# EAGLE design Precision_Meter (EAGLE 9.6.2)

## Sheet 1 of 4: ADC, Buff Amp, VREF Circuits
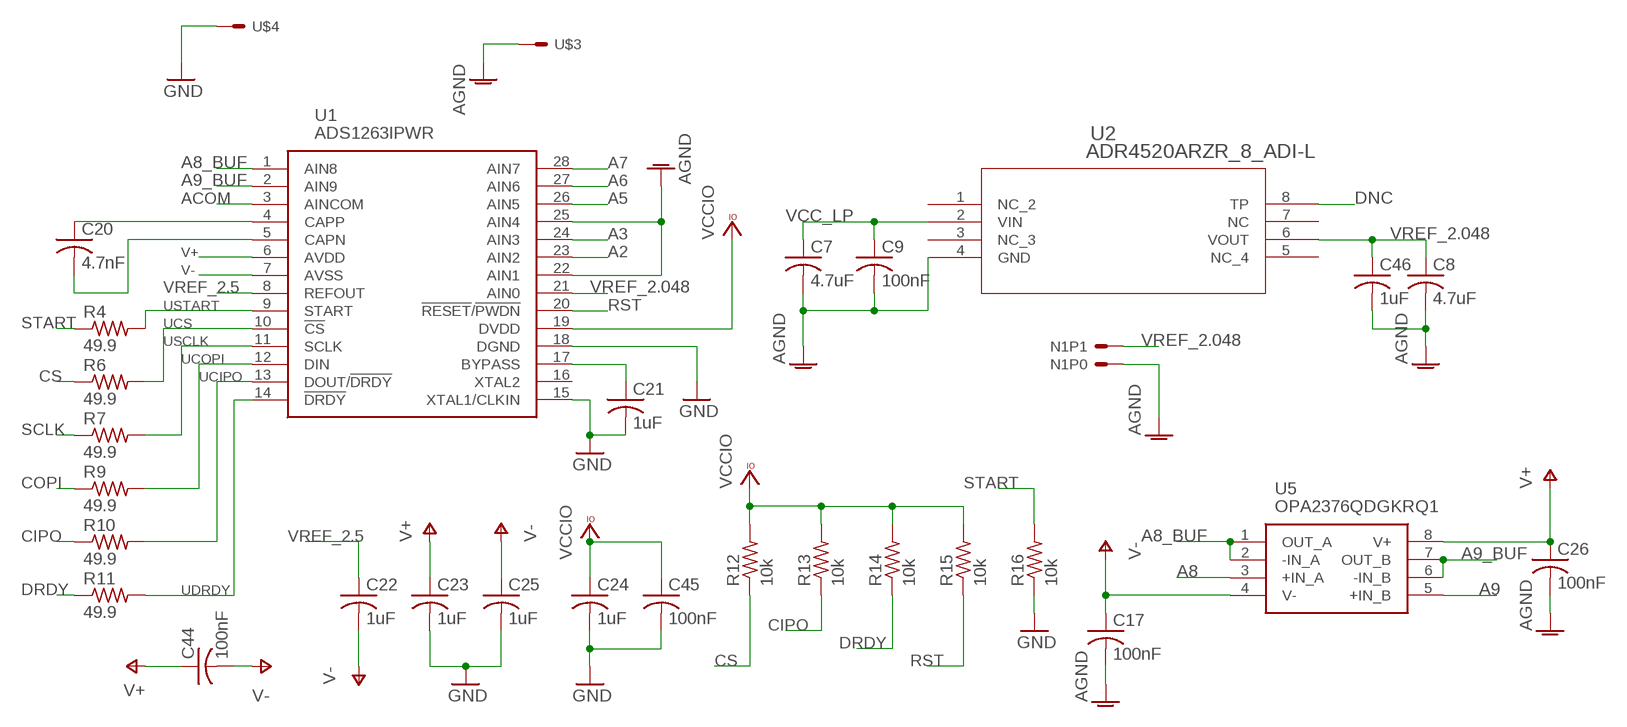
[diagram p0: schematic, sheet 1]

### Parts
C7  4.7uF  C-USC0603  [C0603]
C8  4.7uF  C-USC0603  [C0603]
C9  100nF  C-USC0603  [C0603]
C17  100nF  C-USC0603  [C0603]
C20  4.7nF  C-USC0603  [C0603]
C21  1uF  C-USC0603  [C0603]
C22  1uF  C-USC0603  [C0603]
C23  1uF  C-USC0603  [C0603]
C24  1uF  C-USC0603  [C0603]
C25  1uF  C-USC0603  [C0603]
C26  100nF  C-USC0603  [C0603]
C44  100nF  C-USC0603  [C0603]
C45  100nF  C-USC0603  [C0603]
C46  1uF  C-USC0603  [C0603]
N1  2PINHEADER  [2PINHEADER]
R4  49.9  R-US_R0603  [R0603]
R6  49.9  R-US_R0603  [R0603]
R7  49.9  R-US_R0603  [R0603]
R9  49.9  R-US_R0603  [R0603]
R10  49.9  R-US_R0603  [R0603]
R11  49.9  R-US_R0603  [R0603]
R12  10k  R-US_R0603  [R0603]
R13  10k  R-US_R0603  [R0603]
R14  10k  R-US_R0603  [R0603]
R15  10k  R-US_R0603  [R0603]
R16  10k  R-US_R0603  [R0603]
U1  ADS1263IPWR  [SOP65P640X120-28N]
U2  ADR4520ARZR_8_ADI-L  [R_8_ADI-L]
U5  OPA2376QDGKRQ1  [SOP65P490X110-8N]
U$3  1PINHEADER_S  [1PINHEADER_S]
U$4  1PINHEADER_S  [1PINHEADER_S]

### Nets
A2: U1.23(AIN2) ; also sheet 3
A3: U1.24(AIN3) ; also sheet 3
A5: U1.26(AIN5) ; also sheet 3
A6: U1.27(AIN6) ; also sheet 3
A7: U1.28(AIN7) ; also sheet 3
A8: U5.3(+IN_A) ; also sheet 3
A8_BUF: U1.1(AIN8) U5.1(OUT_A) U5.2(-IN_A)
A9: U5.5(+IN_B) ; also sheet 3
A9_BUF: U1.2(AIN9) U5.6(-IN_B) U5.7(OUT_B)
ACOM: U1.3(AINCOM) ; also sheet 3
AGND: C7.2 C8.2 C9.2 C17.2 C26.2 C46.2 N1.P0 U1.22(AIN1) U1.25(AIN4) U2.4(GND) U$3.P$1(S) ; also sheet 3,4
CIPO: R10.1 R13.1 ; also sheet 3
COPI: R9.1 ; also sheet 3
CS: R6.1 R12.1 ; also sheet 3
DNC: U2.8(TP)
DRDY: R11.1 R14.1 ; also sheet 3
GND: C21.2 C23.2 C24.2 C25.2 C45.2 R16.1 U1.15(XTAL1/CLKIN) U1.18(DGND) U$4.P$1(S) ; also sheet 2,3,4
N$8: C20.1 U1.4(CAPP)
N$9: C20.2 U1.5(CAPN)
N$28: C21.1 U1.17(BYPASS)
RST: R15.1 U1.20(!RESET!/!PWDN) ; also sheet 2,3
SCLK: R7.1 ; also sheet 3
START: R4.1 R16.2 ; also sheet 3
UCIPO: R10.2 U1.13(DOUT/!DRDY)
UCOPI: R9.2 U1.12(DIN)
UCS: R6.2 U1.10(!CS)
UDRDY: R11.2 U1.14(!DRDY)
USCLK: R7.2 U1.11(SCLK)
USTART: R4.2 U1.9(START)
V+: C23.1 C26.1 C44.1 U1.6(AVDD) U5.8(V+) ; also sheet 2
V-: C17.1 C22.2 C25.1 C44.2 U1.7(AVSS) U5.4(V-) ; also sheet 2
VCC_LP: C7.1 C9.1 U2.2(VIN) ; also sheet 2,4
VCCIO: C24.1 C45.1 R12.2 R13.2 R14.2 R15.2 U1.19(DVDD) ; also sheet 2,3
VREF_2.5: C22.1 U1.8(REFOUT)
VREF_2.048: C8.1 C46.1 N1.P1 U1.21(AIN0) U2.6(VOUT)
Unconnected: U1.16(XTAL2) U2.1(NC_2) U2.3(NC_3) U2.5(NC_4) U2.7(NC)

## Sheet 2 of 4: Power Circuits
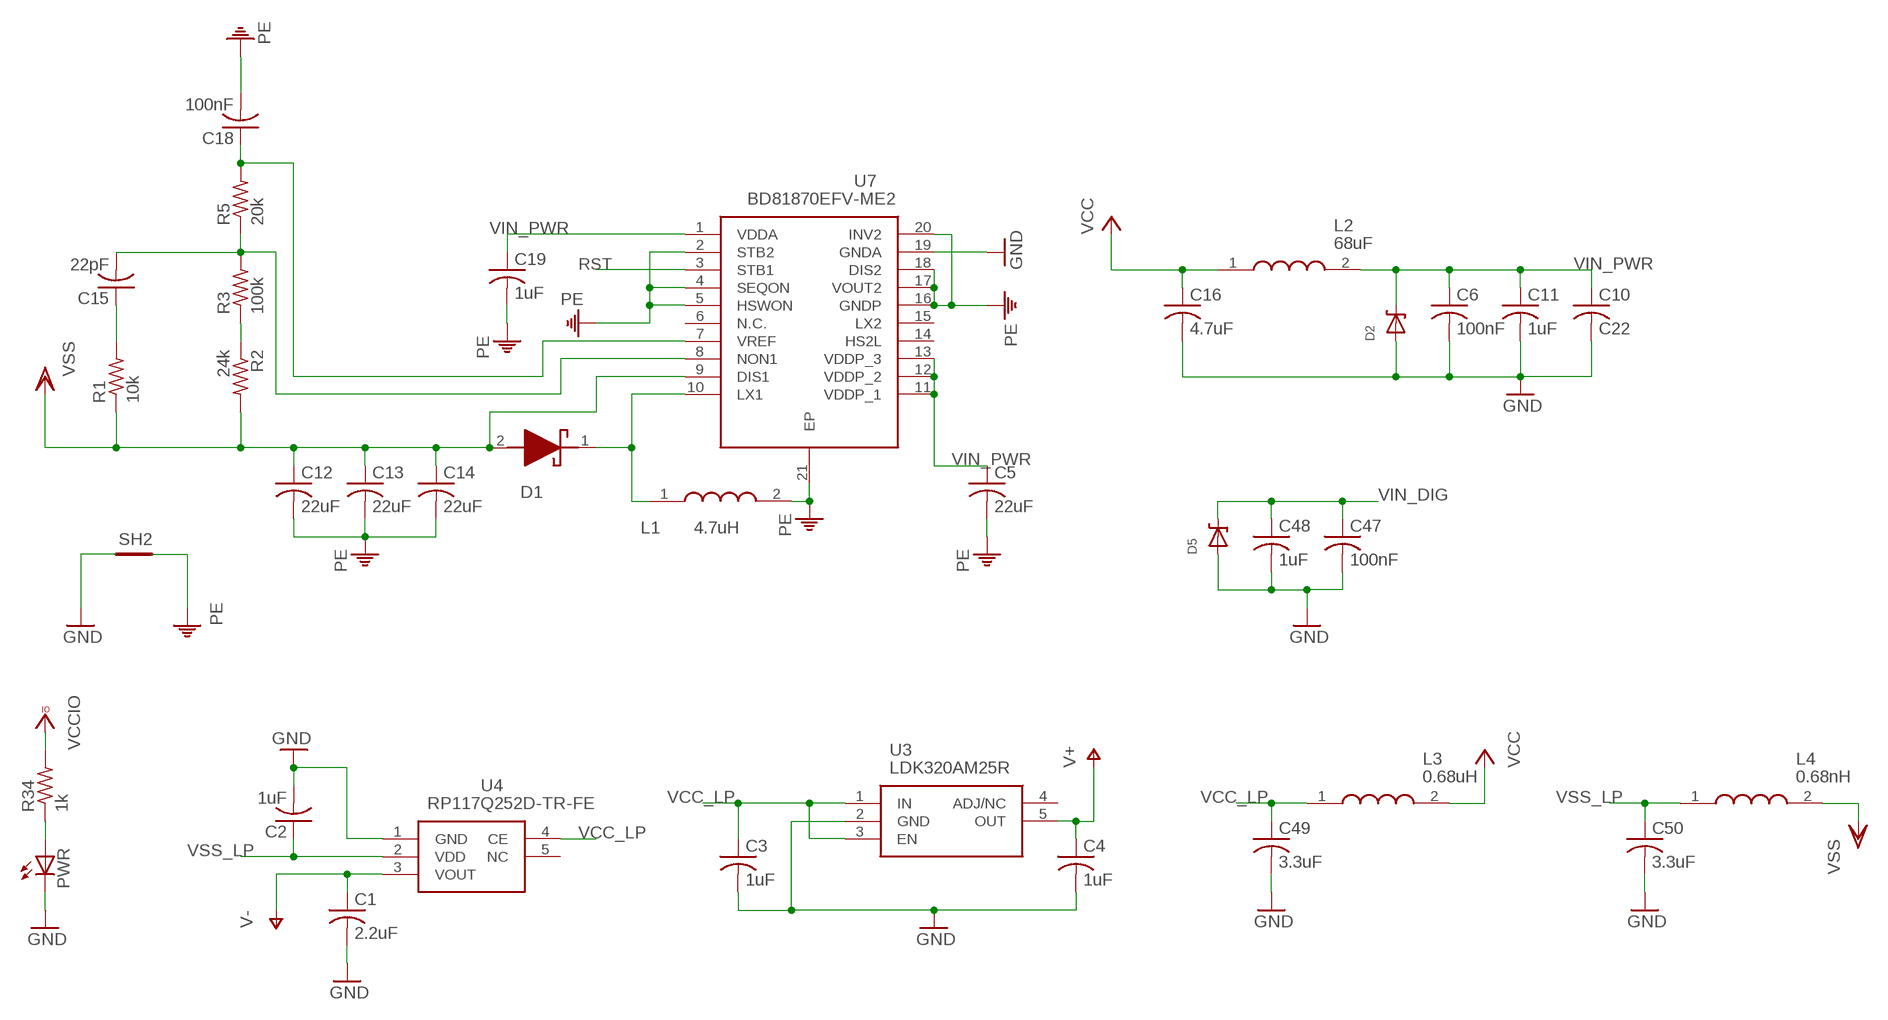
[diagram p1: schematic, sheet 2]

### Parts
C1  2.2uF  C-USC0603  [C0603]
C2  1uF  C-USC0603  [C0603]
C3  1uF  C-USC0603  [C0603]
C4  1uF  C-USC0603  [C0603]
C5  22uF  C-USC0603  [C0603]
C6  100nF  C-USC0603  [C0603]
C10  C22  C-USC0603  [C0603]
C11  1uF  C-USC0603  [C0603]
C12  22uF  C-USC0603  [C0603]
C13  22uF  C-USC0603  [C0603]
C14  22uF  C-USC0603  [C0603]
C15  22pF  C-USC0603  [C0603]
C16  4.7uF  C-USC0603  [C0603]
C18  100nF  C-USC0603  [C0603]
C19  1uF  C-USC0603  [C0603]
C47  100nF  C-USC0603  [C0603]
C48  1uF  C-USC0603  [C0603]
C49  3.3uF  C-USC0603  [C0603]
C50  3.3uF  C-USC0603  [C0603]
D1  RSX051VAM30TR  [RSX051VAM30TR]
D2  DDZ5V6ASF  [DDZ5V6ASF]
D5  DDZ5V6ASF  [DDZ5V6ASF]
L1  4.7uH  LQM21PN4R7MGSD  [LQM21PHR47NG0D]
L2  68uF  LBC3225T680MR  [INDC3225X270N]
L3  0.68uH  MLF2012DR68MT000  [INDC2012X145N]
L4  0.68nH  MLF2012DR68MT000  [INDC2012X145N]
PWR  LEDCHIPLED_0603  [CHIPLED_0603]
R1  10k  R-US_R0603  [R0603]
R2  24k  R-US_R0603  [R0603]
R3  100k  R-US_R0603  [R0603]
R5  20k  R-US_R0603  [R0603]
R34  1k  R-US_R0603  [R0603]
SH2  SHORT-HT5  [SHORT_TOP-50]
U3  LDK320AM25R  [SOT95P280X125-5N]
U4  RP117Q252D-TR-FE  [SOT65P210X110-5N]
U7  BD81870EFV-ME2  [SOP65P640X100-21N]

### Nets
GND: C1.2 C2.2 C3.2 C4.2 C6.2 C10.2 C11.2 C16.2 C47.2 C48.2 C49.2 C50.2 D2.P$1(A) D5.P$1(A) PWR.C SH2.1 U3.2(GND) U4.1(GND) U7.19(GNDA) ; also sheet 1,3,4
N$4: C15.2 R3.2 R5.1 U7.8(NON1)
N$5: D1.1(K) L1.1 U7.10(LX1)
N$6: C18.1 R5.2 U7.7(VREF)
N$7: C15.1 R1.2
N$11: R2.1 R3.1
N$19: PWR.A R34.1
PE: C5.2 C12.2 C13.2 C14.2 C18.2 C19.2 L1.2 SH2.2 U7.2(STB2) U7.4(SEQON) U7.5(HSWON) U7.16(GNDP) U7.17(VOUT2) U7.18(DIS2) U7.20(INV2) U7.21(EP)
RST: U7.3(STB1) ; also sheet 1,3
V+: C4.1 U3.5(OUT) ; also sheet 1
V-: C1.1 U4.3(VOUT) ; also sheet 1
VCC: C16.1 L2.1 L3.2
VCC_LP: C3.1 C49.1 L3.1 U3.1(IN) U3.3(EN) U4.4(CE) ; also sheet 1,4
VCCIO: R34.2 ; also sheet 1,3
VIN_DIG: C47.1 C48.1 D5.P$2(C) ; also sheet 3
VIN_PWR: C5.1 C6.1 C10.1 C11.1 C19.1 D2.P$2(C) L2.2 U7.1(VDDA) U7.11(VDDP_1) U7.12(VDDP_2) U7.13(VDDP_3) ; also sheet 3
VSS: C12.1 C13.1 C14.1 D1.2(A) L4.2 R1.1 R2.2 U7.9(DIS1)
VSS_LP: C2.1 C50.1 L4.1 U4.2(VDD)
Unconnected: U3.4(ADJ/NC) U4.5(NC) U7.6(N.C.) U7.14(HS2L) U7.15(LX2)

## Sheet 3 of 4: Connectors and Switching
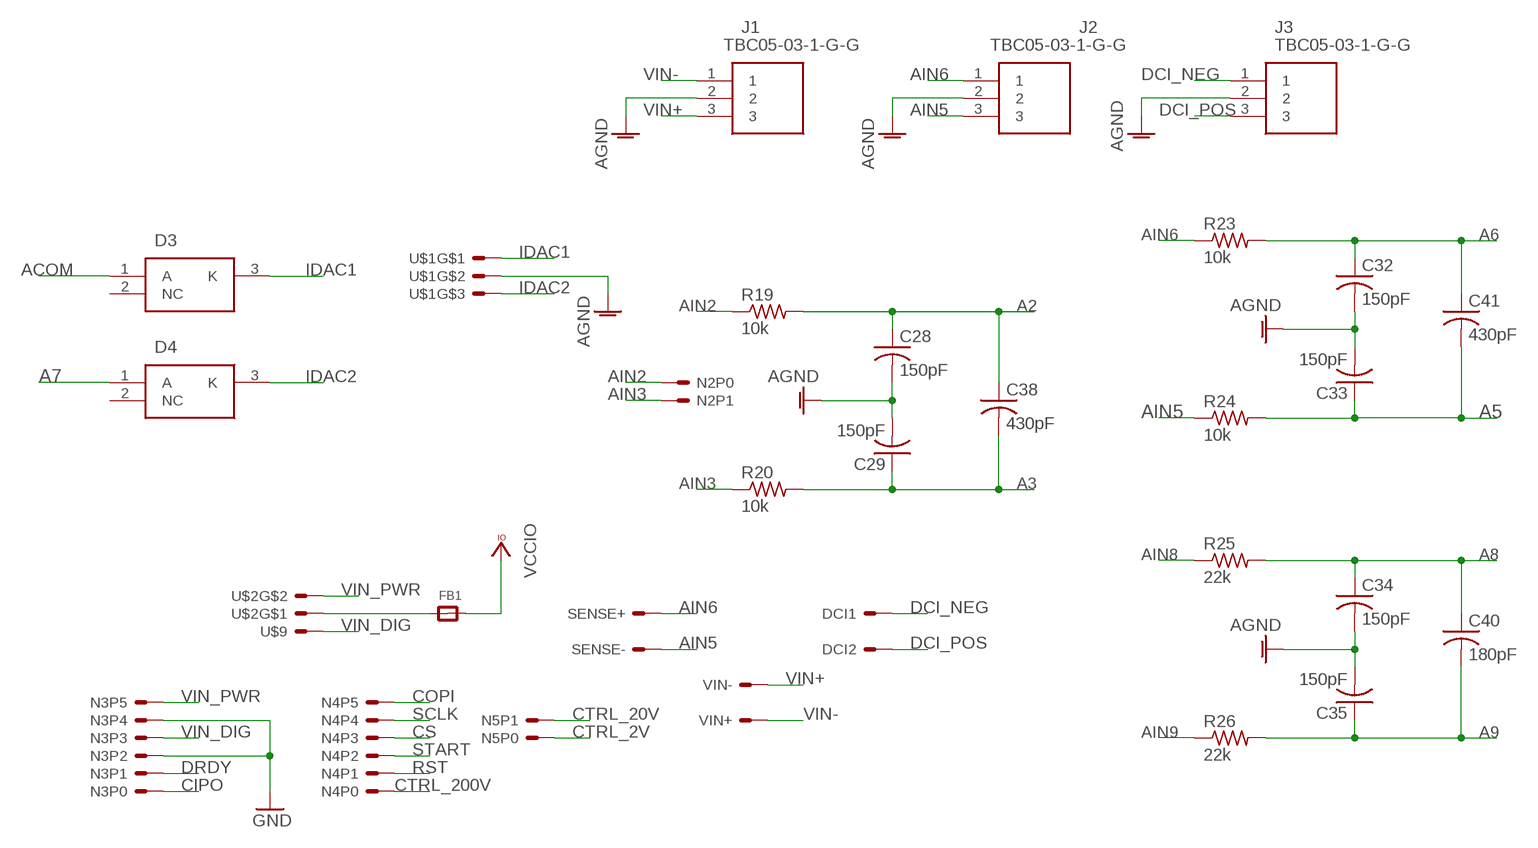
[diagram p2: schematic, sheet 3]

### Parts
C28  150pF  C-USC0603  [C0603]
C29  150pF  C-USC0603  [C0603]
C32  150pF  C-USC0603  [C0603]
C33  150pF  C-USC0603  [C0603]
C34  150pF  C-USC0603  [C0603]
C35  150pF  C-USC0603  [C0603]
C38  430pF  C-USC0603  [C0603]
C40  180pF  C-USC0603  [C0603]
C41  430pF  C-USC0603  [C0603]
D3  BAT54_R1_00001  [SOT95P240X110-3N]
D4  BAT54_R1_00001  [SOT95P240X110-3N]
DCI1  CT3151V1  [CT3151V1]
DCI2  CT3151V1  [CT3151V1]
FB1  FERRITE_0603  [_0603]
J1  TBC05-03-1-G-G  [TBC05031GG]
J2  TBC05-03-1-G-G  [TBC05031GG]
J3  TBC05-03-1-G-G  [TBC05031GG]
N2  2PINHEADER  [2PINHEADER]
N3  6PINHEADER  [6PINHEADER]
N4  6PINHEADER  [6PINHEADER]
N5  2PINHEADER  [2PINHEADER]
R19  10k  R-US_R0603  [R0603]
R20  10k  R-US_R0603  [R0603]
R23  10k  R-US_R0603  [R0603]
R24  10k  R-US_R0603  [R0603]
R25  22k  R-US_R0603  [R0603]
R26  22k  R-US_R0603  [R0603]
SENSE+  CT3151V1  [CT3151V1]
SENSE-  CT3151V1  [CT3151V1]
U$1  3PINHEADER  [3PINHEADER]
U$2  2PINHEADER_S  [2PINHEADER_S]
U$9  1PINHEADER_S  [1PINHEADER_S]
VIN+  CT3151V1  [CT3151V1]
VIN-  CT3151V1  [CT3151V1]

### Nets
A2: C28.1 C38.1 R19.2 ; also sheet 1
A3: C29.1 C38.2 R20.2 ; also sheet 1
A5: C33.1 C41.2 R24.2 ; also sheet 1
A6: C32.1 C41.1 R23.2 ; also sheet 1
A7: D4.1(A) ; also sheet 1
A8: C34.1 C40.1 R25.2 ; also sheet 1
A9: C35.1 C40.2 R26.2 ; also sheet 1
ACOM: D3.1(A) ; also sheet 1
AGND: C28.2 C29.2 C32.2 C33.2 C34.2 C35.2 J1.2 J2.2 J3.2 U$1.N1 ; also sheet 1,4
AIN2: N2.P0 R19.1 ; also sheet 4
AIN3: N2.P1 R20.1 ; also sheet 4
AIN5: J2.3 R24.1 SENSE-.1(S) SENSE-.2(S) SENSE-.3(S) SENSE-.4(S)
AIN6: J2.1 R23.1 SENSE+.1(S) SENSE+.2(S) SENSE+.3(S) SENSE+.4(S)
AIN8: R25.1 ; also sheet 4
AIN9: R26.1 ; also sheet 4
CIPO: N3.P0 ; also sheet 1
COPI: N4.P5 ; also sheet 1
CS: N4.P3 ; also sheet 1
CTRL_2V: N5.P0 ; also sheet 4
CTRL_20V: N5.P1 ; also sheet 4
CTRL_200V: N4.P0 ; also sheet 4
DCI_NEG: DCI1.1(S) DCI1.2(S) DCI1.3(S) DCI1.4(S) J3.1 ; also sheet 4
DCI_POS: DCI2.1(S) DCI2.2(S) DCI2.3(S) DCI2.4(S) J3.3 ; also sheet 4
DRDY: N3.P1 ; also sheet 1
GND: N3.P2 N3.P4 ; also sheet 1,2,4
IDAC1: D3.3(K) U$1.N0
IDAC2: D4.3(K) U$1.N2
N$17: FB1.1 U$2.N0
RST: N4.P1 ; also sheet 1,2
SCLK: N4.P4 ; also sheet 1
START: N4.P2 ; also sheet 1
VCCIO: FB1.2 ; also sheet 1,2
VIN+: J1.3 VIN-.1(S) VIN-.2(S) VIN-.3(S) VIN-.4(S) ; also sheet 4
VIN-: J1.1 VIN+.1(S) VIN+.2(S) VIN+.3(S) VIN+.4(S) ; also sheet 4
VIN_DIG: N3.P3 U$9.P$1(S) ; also sheet 2
VIN_PWR: N3.P5 U$2.N1 ; also sheet 2
Unconnected: D3.2(NC) D4.2(NC)

## Sheet 4 of 4: Meter Front End
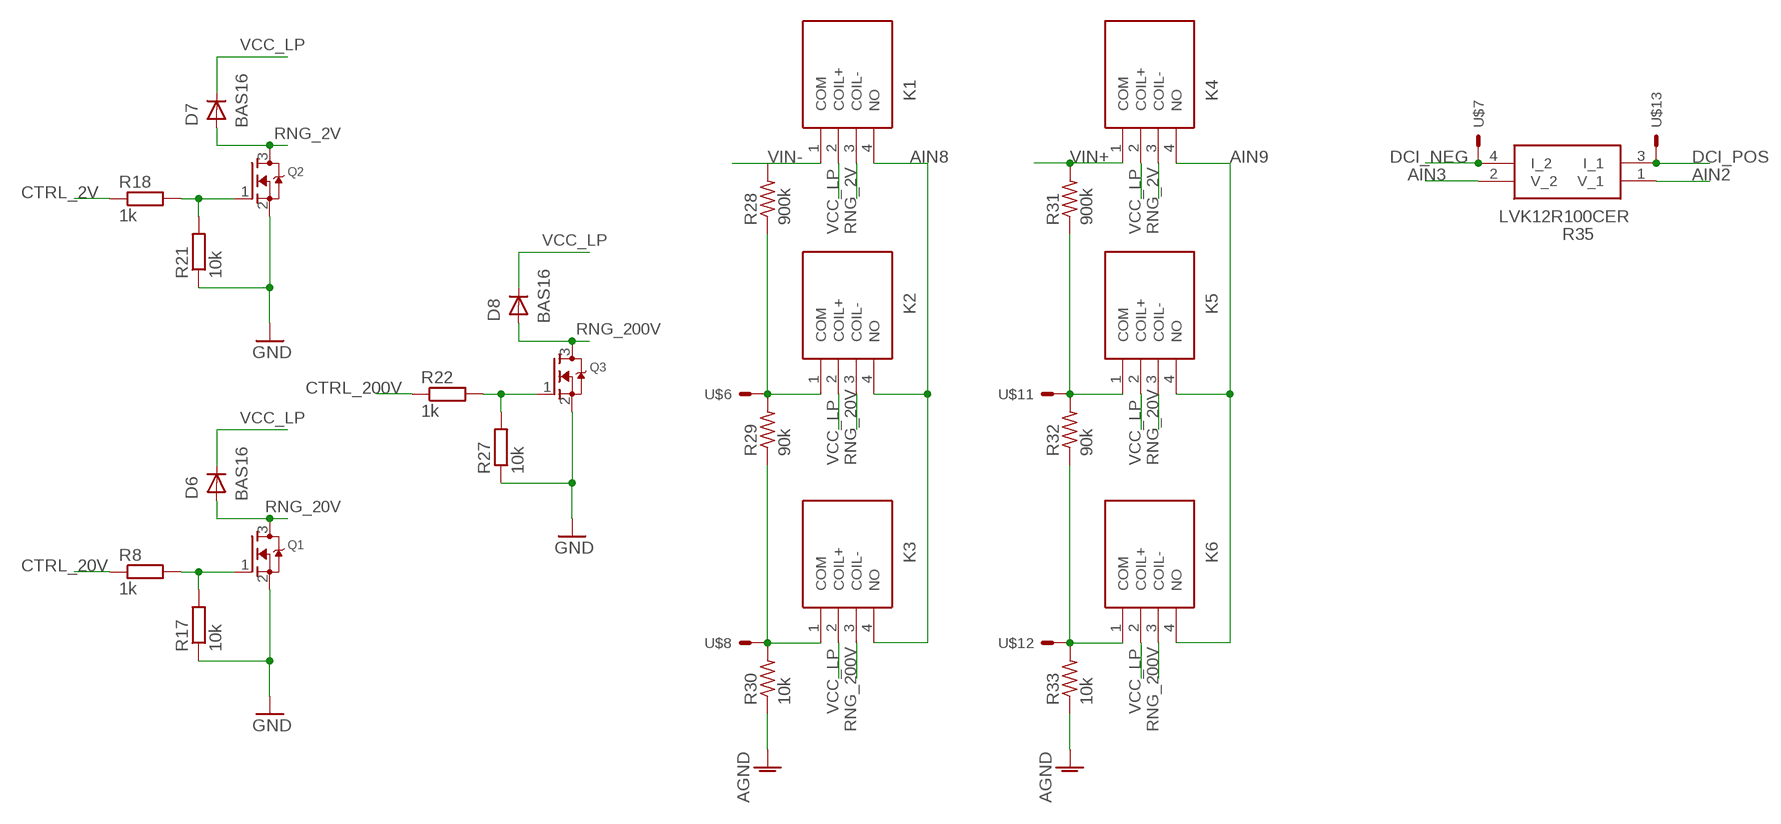
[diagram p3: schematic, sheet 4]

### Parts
D6  BAS16  [SOT23]
D7  BAS16  [SOT23]
D8  BAS16  [SOT23]
K1  HE3621A0500  [HE3621A0500]
K2  HE3621A0500  [HE3621A0500]
K3  HE3621A0500  [HE3621A0500]
K4  HE3621A0500  [HE3621A0500]
K5  HE3621A0500  [HE3621A0500]
K6  HE3621A0500  [HE3621A0500]
Q1  MOSFET-NREFLOW  [SOT23-R]
Q2  MOSFET-NREFLOW  [SOT23-R]
Q3  MOSFET-NREFLOW  [SOT23-R]
R8  1k  R-EU_R0603  [R0603]
R17  10k  R-EU_R0603  [R0603]
R18  1k  R-EU_R0603  [R0603]
R21  10k  R-EU_R0603  [R0603]
R22  1k  R-EU_R0603  [R0603]
R27  10k  R-EU_R0603  [R0603]
R28  900k  R-US_R1206  [R1206]
R29  90k  R-US_R1206  [R1206]
R30  10k  R-US_R0603  [R0603]
R31  900k  R-US_R1206  [R1206]
R32  90k  R-US_R1206  [R1206]
R33  10k  R-US_R0603  [R0603]
R35  LVK12R100CER  [LVK12R100CER]
U$6  1PINHEADER_S  [1PINHEADER_S]
U$7  1PINHEADER_S  [1PINHEADER_S]
U$8  1PINHEADER_S  [1PINHEADER_S]
U$11  1PINHEADER_S  [1PINHEADER_S]
U$12  1PINHEADER_S  [1PINHEADER_S]
U$13  1PINHEADER_S  [1PINHEADER_S]

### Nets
AGND: R30.1 R33.1 ; also sheet 1,3
AIN2: R35.1(V_1) ; also sheet 3
AIN3: R35.2(V_2) ; also sheet 3
AIN8: K1.4(NO) K2.4(NO) K3.4(NO) ; also sheet 3
AIN9: K4.4(NO) K5.4(NO) K6.4(NO) ; also sheet 3
CTRL_2V: R18.1 ; also sheet 3
CTRL_20V: R8.1 ; also sheet 3
CTRL_200V: R22.1 ; also sheet 3
DCI_NEG: R35.4(I_2) U$7.P$1(S) ; also sheet 3
DCI_POS: R35.3(I_1) U$13.P$1(S) ; also sheet 3
GND: Q1.2(S) Q2.2(S) Q3.2(S) R17.1 R21.1 R27.1 ; also sheet 1,2,3
N$2: Q1.1(G) R8.2 R17.2
N$10: K2.1(COM) R28.1 R29.2 U$6.P$1(S)
N$12: K3.1(COM) R29.1 R30.2 U$8.P$1(S)
N$14: K5.1(COM) R31.1 R32.2 U$11.P$1(S)
N$16: K6.1(COM) R32.1 R33.2 U$12.P$1(S)
N$22: Q2.1(G) R18.2 R21.2
N$25: Q3.1(G) R22.2 R27.2
RNG_2V: D7.1(A) K1.3(COIL-) K4.3(COIL-) Q2.3(D)
RNG_20V: D6.1(A) K2.3(COIL-) K5.3(COIL-) Q1.3(D)
RNG_200V: D8.1(A) K3.3(COIL-) K6.3(COIL-) Q3.3(D)
VCC_LP: D6.3(K) D7.3(K) D8.3(K) K1.2(COIL+) K2.2(COIL+) K3.2(COIL+) K4.2(COIL+) K5.2(COIL+) K6.2(COIL+) ; also sheet 1,2
VIN+: K4.1(COM) R31.2 ; also sheet 3
VIN-: K1.1(COM) R28.2 ; also sheet 3

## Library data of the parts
C1-C26 C28 C29 C32-C35 C38 C40 C41 C44-C50 = rcl:C-US: CAPACITOR, American symbol; SPICEPREFIX: C
D1 = SamacSys_Parts:RSX051VAM30TR: ROHM 30V 500mA, SiC Schottky Diode, 2-Pin SOD-323HE RSX051VAM30TR; DESCRIPTION: ROHM 30V 500mA, SiC Schottky Diode, 2-Pin SOD-323HE RSX051VAM30TR; HEIGHT: 0.8mm; MANUFACTURER_NAME: ROHM Semiconductor; MANUFACTURER_PART_NUMBER: RSX051VAM30TR; MOUSER_PART_NUMBER: 755-RSX051VAM30TR; MOUSER_PRICE-STOCK: https://www.mouser.co.uk/ProductDetail/ROHM-Semiconductor/RSX051VAM30TR?qs=4v%252BiZTmLVHH6gyykIHF0SA%3D%3D
D2 D5 = ForceTronics:DDZ5V6ASF: DDZ5V6ASF 5.42 Zener Diode
D3 D4 = SamacSys_Parts:BAT54_R1_00001: Diode 30V 200mA Surface Mount SOT-23 Source: Datasheet; DESCRIPTION: Diode 30V 200mA Surface Mount SOT-23; HEIGHT: 1.1mm; MANUFACTURER_NAME: PANJIT; MANUFACTURER_PART_NUMBER: BAT54_R1_00001; MOUSER_PART_NUMBER: 241-BAT54_R1_00001; MOUSER_PRICE-STOCK: https://www.mouser.co.uk/ProductDetail/Panjit/BAT54_R1_00001?qs=sPbYRqrBIVlJNaHalS0dJg%3D%3D
D6-D8 = nxp_60:BAS16: High-speed switching diode
DCI1 DCI2 SENSE+ SENSE- VIN+ VIN- = ForceTronics:CT3151V1: Device footprint for PCB mount straight banana connector. One connection point, but four through hole pins
FB1 = microbuilder:FERRITE: Ferrite Bead
J1-J3 = SamacSys_Parts:TBC05-03-1-G-G: 3 Position Wire to Board Terminal Block Horizontal with Board 0.100" (2.54mm) Through Hole Source: Datasheet; DESCRIPTION: 3 Position Wire to Board Terminal Block Horizontal with Board 0.100" (2.54mm) Through Hole; HEIGHT: 8.8mm; MANUFACTURER_NAME: GCT (GLOBAL CONNECTOR TECHNOLOGY); MANUFACTURER_PART_NUMBER: TBC05-03-1-G-G
K1-K6 = SamacSys_Parts:HE3621A0500: RELAY REED SPST 500MA 5V Source: Datasheet; DESCRIPTION: RELAY REED SPST 500MA 5V; HEIGHT: 7mm; MANUFACTURER_NAME: LITTELFUSE; MANUFACTURER_PART_NUMBER: HE3621A0500; MOUSER_PART_NUMBER: 934-HE3621A0500; MOUSER_PRICE-STOCK: https://www.mouser.co.uk/ProductDetail/Littelfuse/HE3621A0500?qs=X8LBAgEWIKIc9wEjZ29LbA%3D%3D
L1 = SamacSys_Parts:LQM21PN4R7MGSD: LQM21PN_GS Series Inductor 4.7uH +/-20% 0805 (2012); DESCRIPTION: LQM21PN_GS Series Inductor 4.7uH +/-20% 0805 (2012); HEIGHT: 1mm; MANUFACTURER_NAME: Murata Electronics; MANUFACTURER_PART_NUMBER: LQM21PN4R7MGSD; MOUSER_PART_NUMBER: 81-LQM21PN4R7MGSD; MOUSER_PRICE-STOCK: https://www.mouser.co.uk/ProductDetail/Murata-Electronics/LQM21PN4R7MGSD?qs=Gufeu08L%2Fl2uzbzo%2FrY4bg%3D%3D
L2 = SamacSys_Parts:LBC3225T680MR: Power Inductors - SMD 963-LSQCA322525T680M RPLCMT PN 1210 68uH 1300mOhms 190mA; DESCRIPTION: Power Inductors - SMD 963-LSQCA322525T680M RPLCMT PN 1210 68uH 1300mOhms 190mA; HEIGHT: 2.7mm; MANUFACTURER_NAME: TAIYO YUDEN; MANUFACTURER_PART_NUMBER: LBC3225T680MR; MOUSER_PART_NUMBER: 963-LBC3225T680MR; MOUSER_PRICE-STOCK: https://www.mouser.co.uk/ProductDetail/Taiyo-Yuden/LBC3225T680MR?qs=PzICbMaShUfaVZGcpQe%2FGA%3D%3D
L3 L4 = SamacSys_Parts:MLF2012DR68MT000: SMD / SMT Inductors (Coils), L=0.68?H, L x W x T :; DESCRIPTION: SMD / SMT Inductors (Coils), L=0.68?H, L x W x T :; HEIGHT: 1.45mm; MANUFACTURER_NAME: TDK; MANUFACTURER_PART_NUMBER: MLF2012DR68MT000
N1 N2 N5 = ForceTronics:2PINHEADER
N3 N4 = ForceTronics-ForceTronics:6PINHEADER
PWR = adafruit:LED: LED
Q1-Q3 = microbuilder:MOSFET-N: N-Channel Mosfet LEGEND VDS: Voltage Drain-Source ID: Drain Current RDS(ON): Drain-Source On-State Resistance VGS(TH): Gate-Source Threshold Voltage CISS: Drain-Source Input Capacitance SOT-23 Name VDS ID RDS(ON) VGS(TH) CISS Order Number 2N7002E 60V 260mA 2.5 Ohm 2.5V @ 250uA 26.7pF @ 25V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
R1-R7 R9-R16 R19 R20 R23-R26 R28-R34 = rcl:R-US_: RESISTOR, American symbol; SPICEPREFIX: R
R8 R17 R18 R21 R22 R27 = rcl:R-EU_: RESISTOR, European symbol; SPICEPREFIX: R
R35 = SamacSys_Parts:LVK12R100CER: Current Sense Resistors - SMD .1 OHM.25% 1/2W Source: Datasheet; DESCRIPTION: Current Sense Resistors - SMD .1 OHM.25% 1/2W; HEIGHT: 0.65mm; MANUFACTURER_NAME: Ohmite; MANUFACTURER_PART_NUMBER: LVK12R100CER; MOUSER_PART_NUMBER: 588-LVK12R100CER; MOUSER_PRICE-STOCK: https://www.mouser.co.uk/ProductDetail/Ohmite/LVK12R100CER?qs=Cb2nCFKsA8oBVfMdwpyWoQ%3D%3D
SH2 = shorts-old:SHORT-H: Short between two nets; BOM: no
U1 = SamacSys_Parts:ADS1263IPWR: 32-Bit, 38kSPS, 10-Ch Delta-Sigma ADC w/ PGA, Voltage Reference, and Aux ADC for Factory Automation Source: Datasheet; DESCRIPTION: 32-Bit, 38kSPS, 10-Ch Delta-Sigma ADC w/ PGA, Voltage Reference, and Aux ADC for Factory Automation; HEIGHT: 1.2mm; MANUFACTURER_NAME: Texas Instruments; MANUFACTURER_PART_NUMBER: ADS1263IPWR; MOUSER_PART_NUMBER: 595-ADS1263IPWR; MOUSER_PRICE-STOCK: https://www.mouser.co.uk/ProductDetail/Texas-Instruments/ADS1263IPWR?qs=GURawfaeGuAEKG2KPkczsw%3D%3D
U2 = ForceTronics:ADR4520ARZ; COPYRIGHT: Copyright (C) 2025 Ultra Librarian. All rights reserved.; MANUFACTURER_PART_NUMBER: ADR4520ARZ; MFR_NAME: Analog Devices Inc
U3 = SamacSys_Parts:LDK320AM25R: 200 mA low quiescent current and high PSRR voltage regulator Source: Datasheet; DESCRIPTION: 200 mA low quiescent current and high PSRR voltage regulator; HEIGHT: 1.25mm; MANUFACTURER_NAME: STMicroelectronics; MANUFACTURER_PART_NUMBER: LDK320AM25R; MOUSER_PART_NUMBER: 511-LDK320AM25R; MOUSER_PRICE-STOCK: https://www.mouser.co.uk/ProductDetail/STMicroelectronics/LDK320AM25R?qs=wd5RIQLrsJiQNxEkfV2I5w%3D%3D
U4 = SamacSys_Parts:RP117Q252D-TR-FE: LDO Voltage Regulators 100 mA LDO Regulator Source: Datasheet; DESCRIPTION: LDO Voltage Regulators 100 mA LDO Regulator; HEIGHT: 1.1mm; MANUFACTURER_NAME: Nisshinbo; MANUFACTURER_PART_NUMBER: RP117Q252D-TR-FE; MOUSER_PART_NUMBER: 848-RP117Q252D-TR-FE; MOUSER_PRICE-STOCK: https://www.mouser.co.uk/ProductDetail/Nisshinbo/RP117Q252D-TR-FE?qs=0lQeLiL1qyb%252B39Gkjsmryg%3D%3D
U5 = SamacSys_Parts:OPA2376QDGKRQ1: Low Noise, Low Quiescent Current, Precision Operational Amplifier e-trim/trade Source: Datasheet; DESCRIPTION: Low Noise, Low Quiescent Current, Precision Operational Amplifier e-trim/trade; HEIGHT: 1.1mm; MANUFACTURER_NAME: Texas Instruments; MANUFACTURER_PART_NUMBER: OPA2376QDGKRQ1; MOUSER_PART_NUMBER: 595-OPA2376QDGKRQ1; MOUSER_PRICE-STOCK: https://www.mouser.co.uk/ProductDetail/Texas-Instruments/OPA2376QDGKRQ1?qs=zEmsApcVOkU338m46%2F1O7A%3D%3D
U7 = SamacSys_Parts:BD81870EFV-ME2: ROHM - BD81870EFV-ME2 - DC/DC Switching Regulator, Inverting, Step Up, 2 Output, 2.5V to 5.5VIn, 18V out, 2.1MHz, HTSSOP-20 Source: Datasheet; DESCRIPTION: ROHM - BD81870EFV-ME2 - DC/DC Switching Regulator, Inverting, Step Up, 2 Output, 2.5V to 5.5VIn, 18V out, 2.1MHz, HTSSOP-20; HEIGHT: 1mm; MANUFACTURER_NAME: ROHM Semiconductor; MANUFACTURER_PART_NUMBER: BD81870EFV-ME2; MOUSER_PART_NUMBER: 755-BD81870EFV-ME2; MOUSER_PRICE-STOCK: https://www.mouser.co.uk/ProductDetail/ROHM-Semiconductor/BD81870EFV-ME2/?qs=HXFqYaX1Q2wm5IkeUd4YKg%3D%3D
U$1 = ForceTronics:3PINHEADER: 3 pin header with oval copper
U$2 = ForceTronics:2PINHEADER_S: 2 pin header with round copper
U$3 U$4 = ForceTronics-ForceTronics:1PINHEADER_S: 1 pin header with round pad
U$6-U$9 U$11-U$13 = ForceTronics:1PINHEADER_S: 1 pin header with round pad

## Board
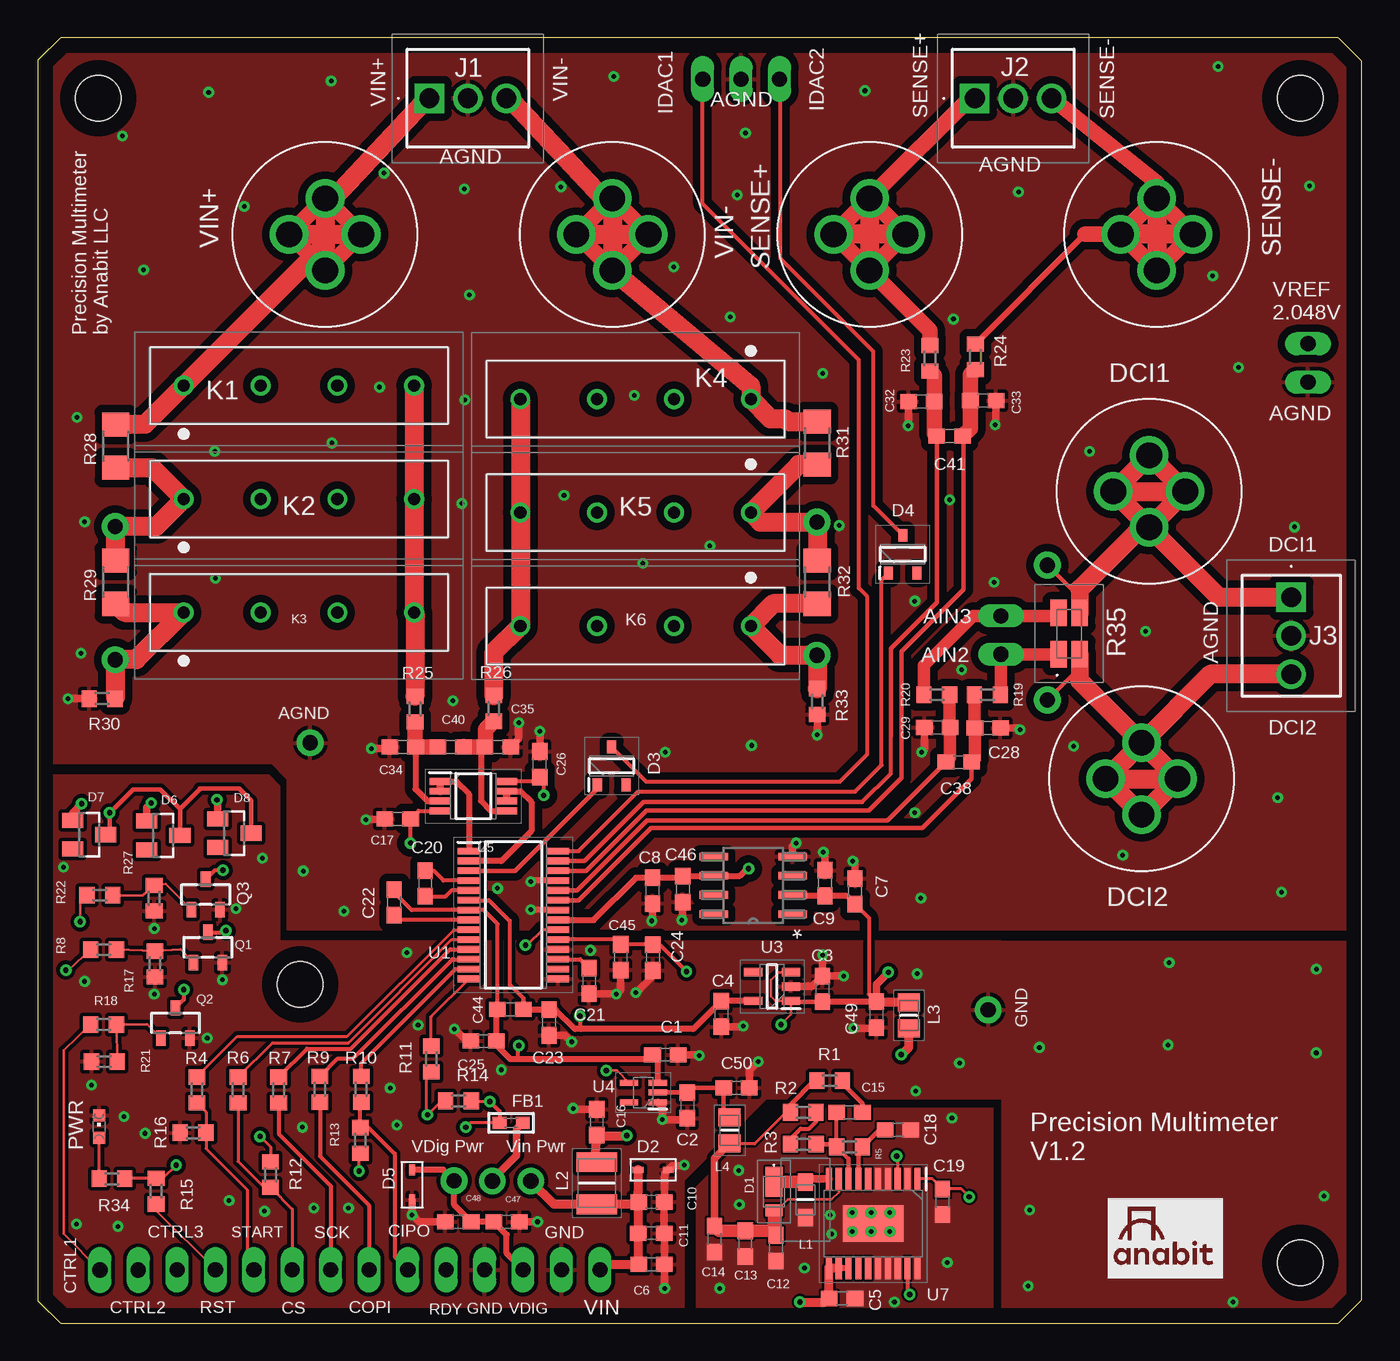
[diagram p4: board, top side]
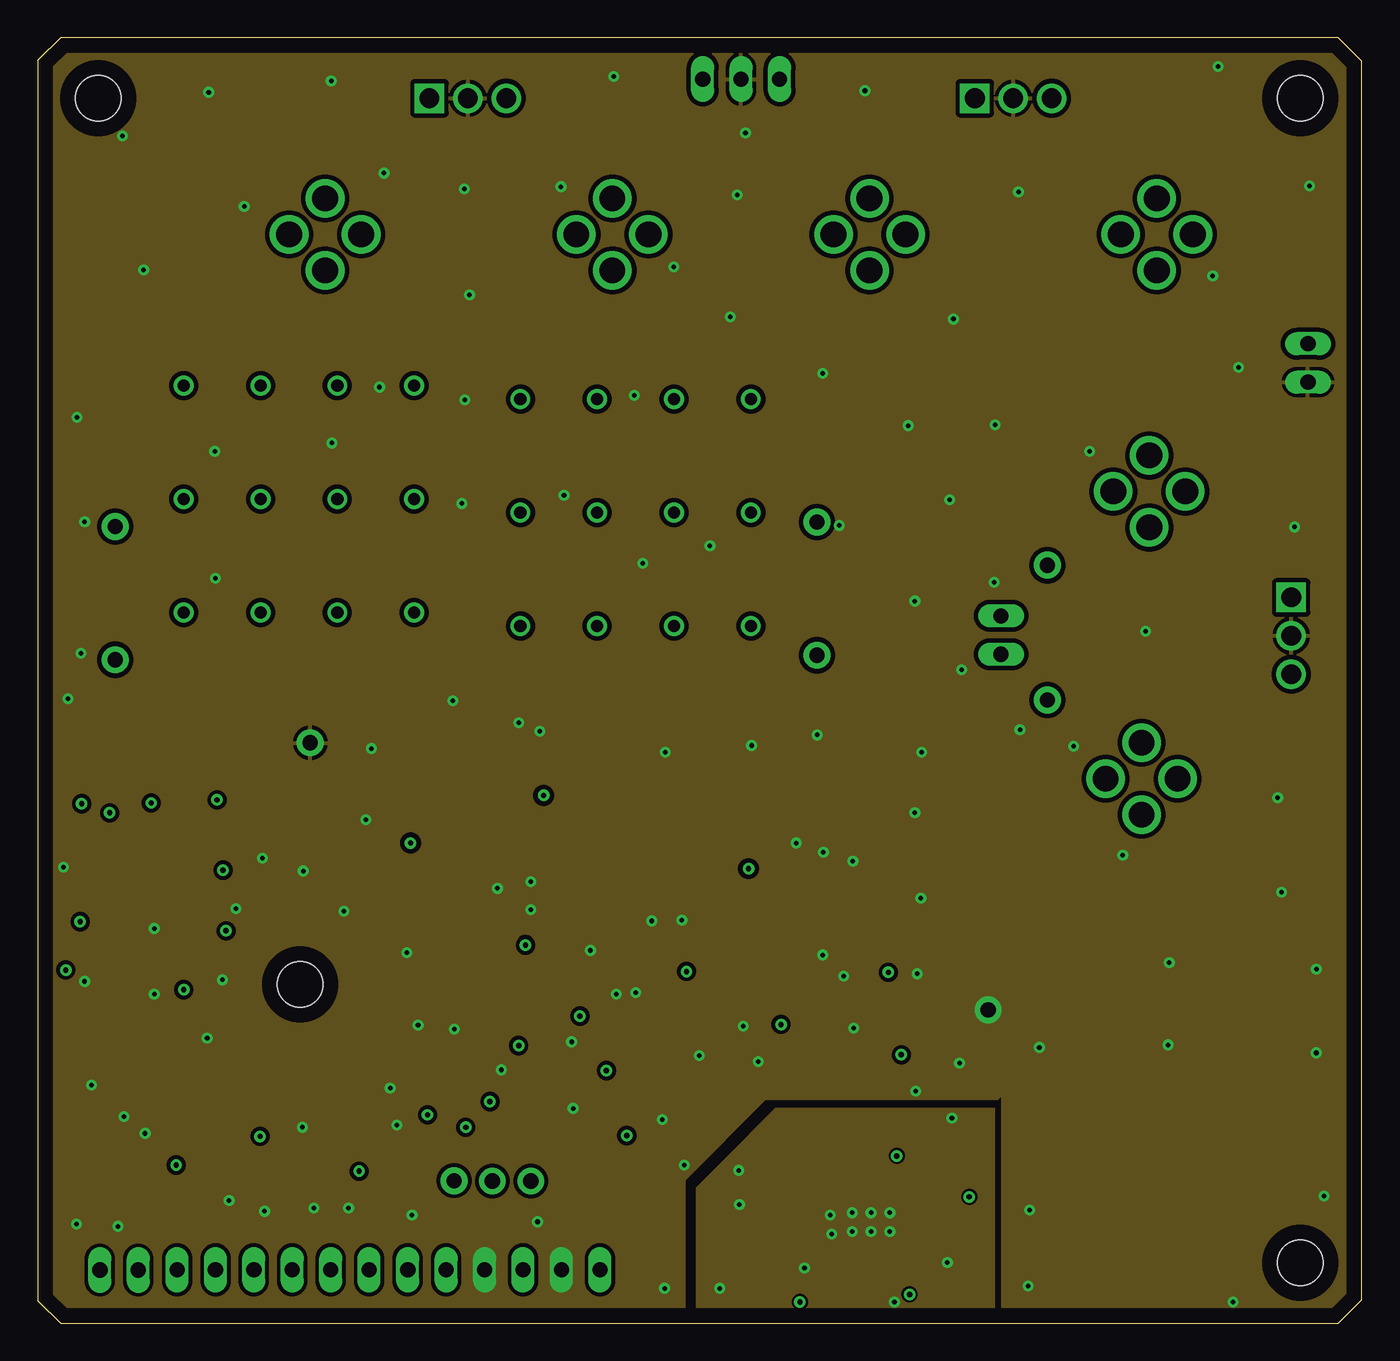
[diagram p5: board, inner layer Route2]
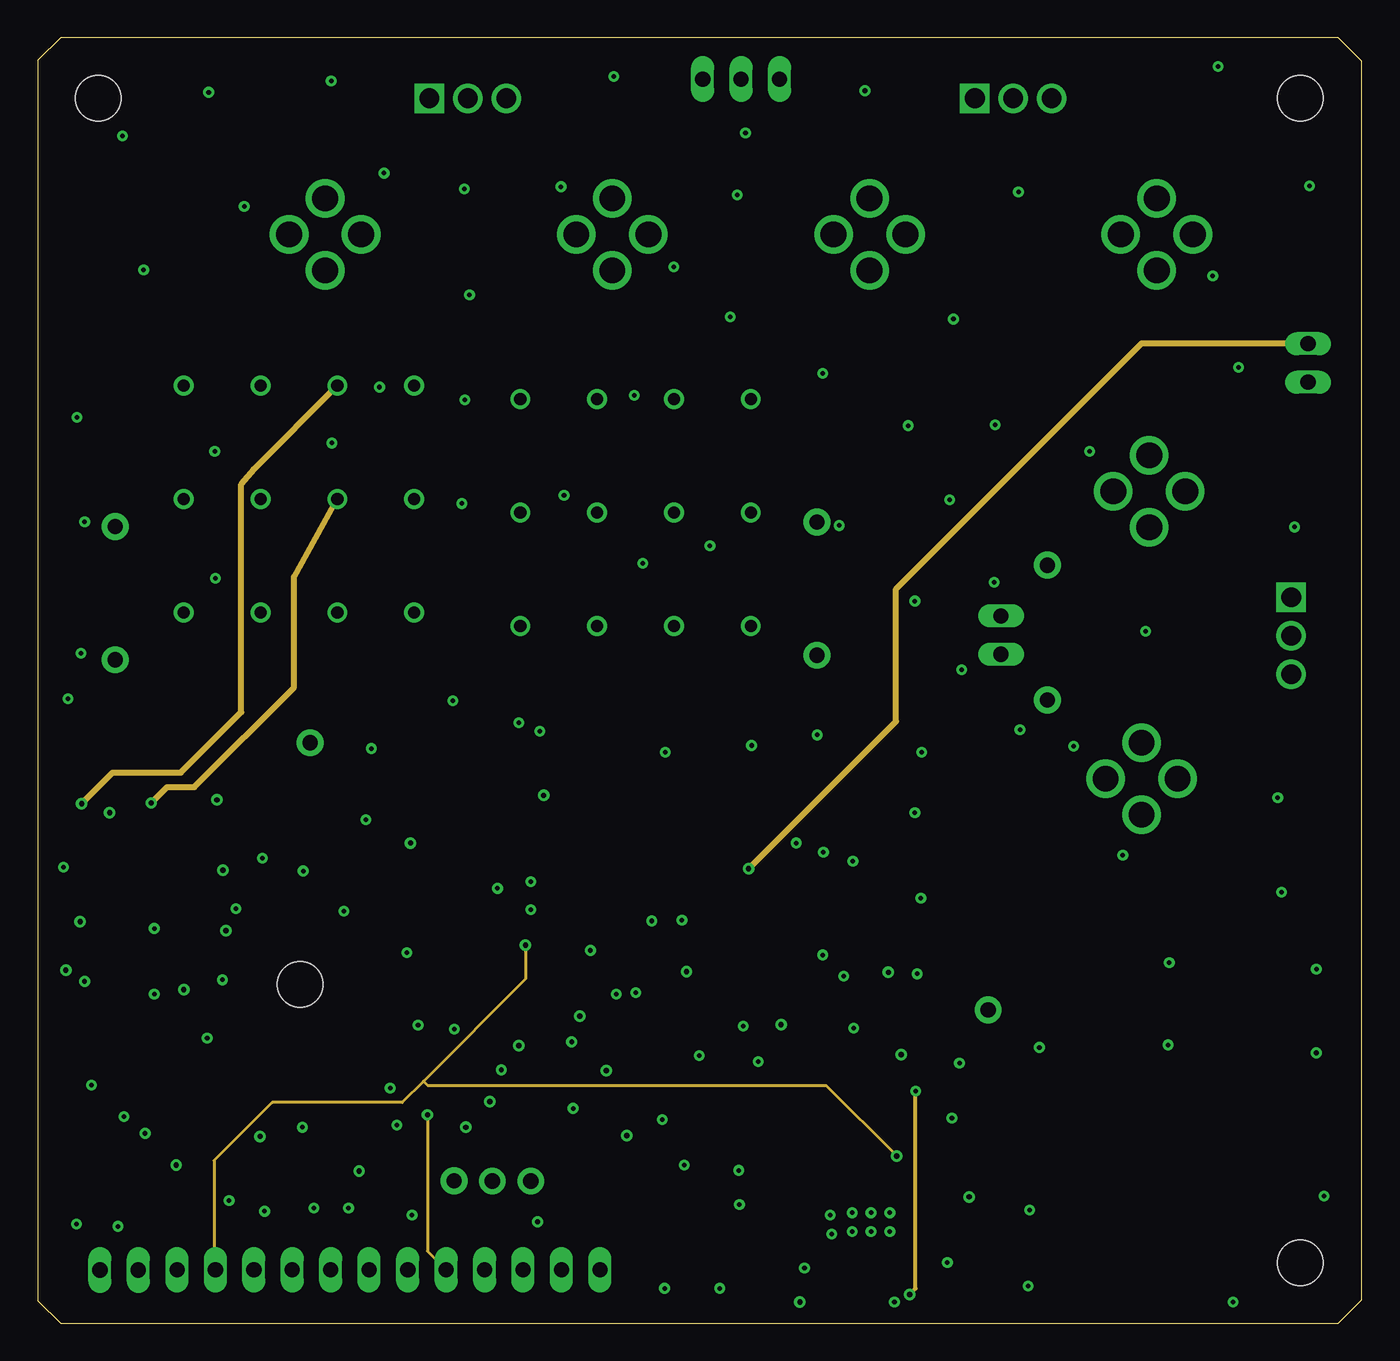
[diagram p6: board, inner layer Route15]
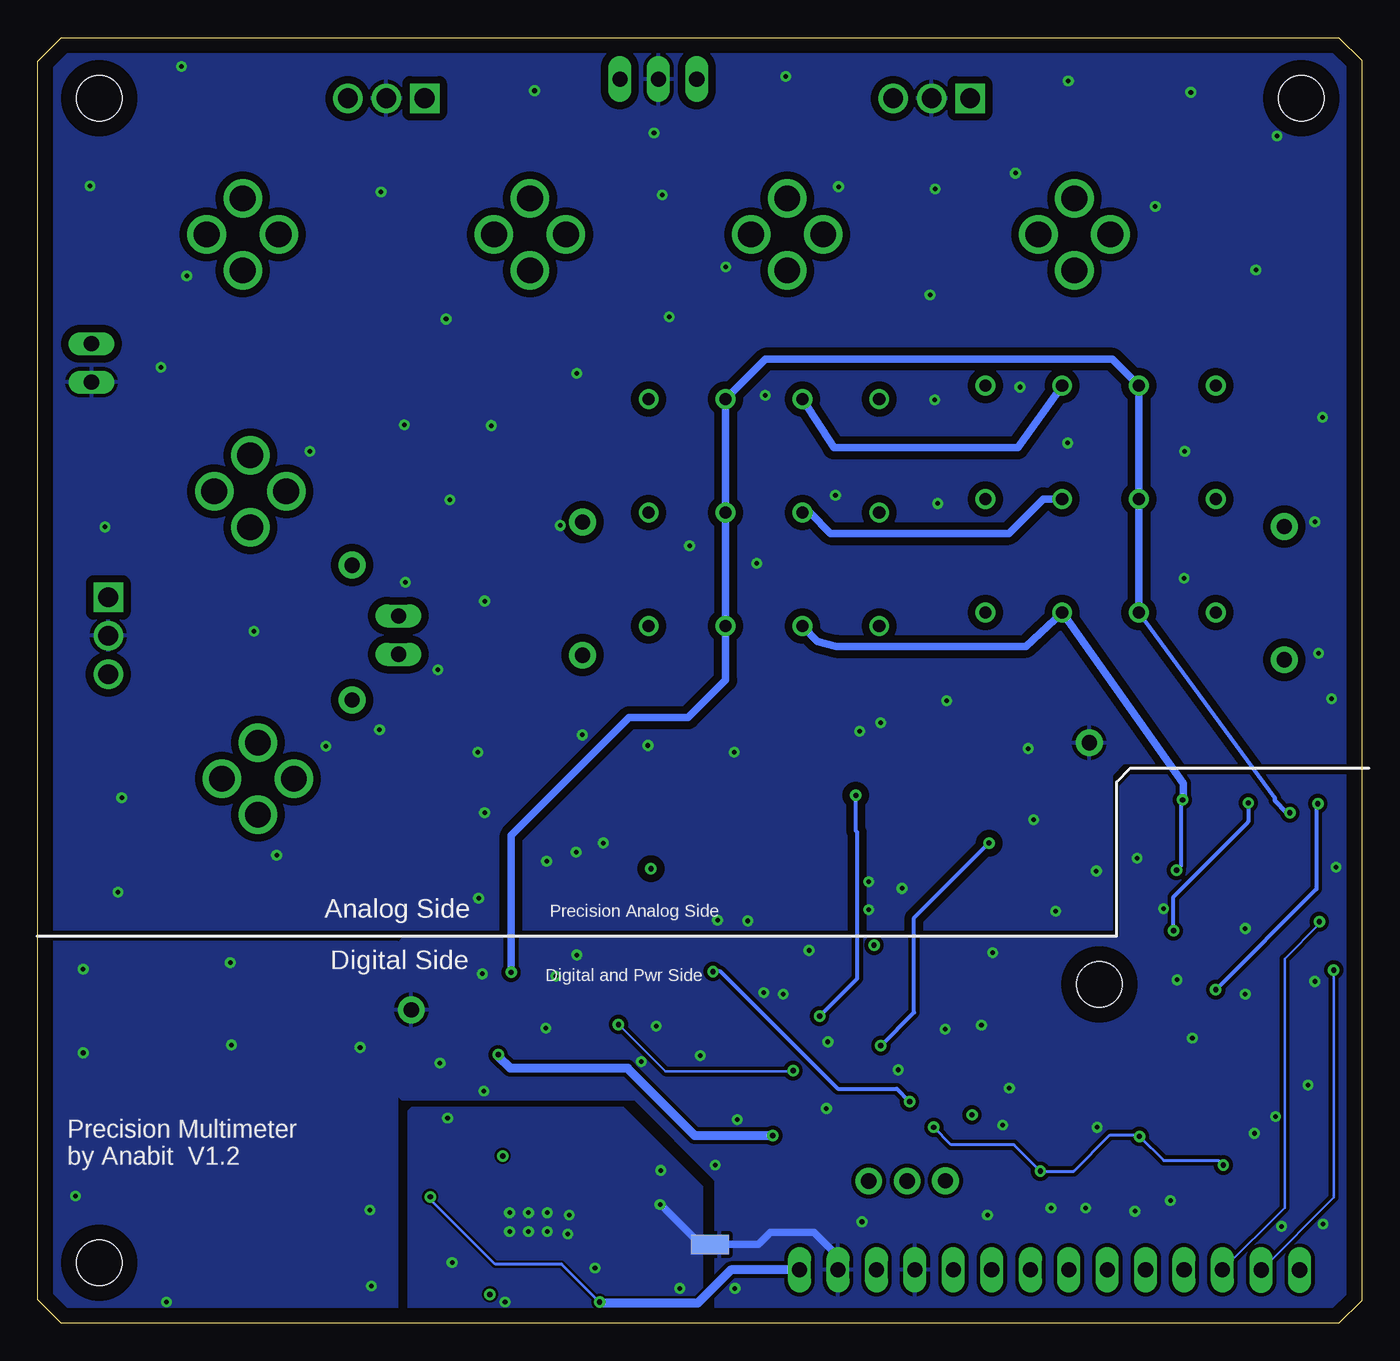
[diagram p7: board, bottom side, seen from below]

Size 87.55 x 85 mm. Coordinates in mm from the lower left corner, seen from the top.
Outline: 1.5,0 86,0 87.55,1.55 87.54,83.46 86.01,85 1.5,85 0,83.51 0.01,1.49 1.5,0
Copper layers (1+2*15+16): Top 0.035mm / dielectric 0.5mm / Route2 0.035mm / dielectric 0.75mm / Route15 0.035mm / dielectric 0.75mm / Bottom 0.035mm
Design rules "default *": minimum track width 6mil, minimum drill 0.3mm, track to track 6mil, track to pad 6mil, pad to pad 6mil, via to via 6mil, smd to smd 6mil, copper to edge 40mil, drill to drill 6mil, minimum pad ring 10mil, minimum via ring 8mil, stop-mask expansion 4mil, vias tented up to drill 0mil, thermal gap 10mil
Holes 3 mm at 83.5,81 4,81 17.35,22.4 83.5,4

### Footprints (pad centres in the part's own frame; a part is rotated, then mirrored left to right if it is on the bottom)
C0603 = smd 1.1 x 1: 1 -0.85,0; 2 0.85,0
RSX051VAM30TR = smd 1.1 x 2: 1 0,0.65 | smd 1.1 x 0.8: 2 0,-1.25
DDZ5V6ASF = smd 0.71 x 0.41: P$1 0,0; P$2 1.99,0
SOT95P240X110-3N = smd 0.85 x 0.6: 1 -1.25,0.95; 2 -1.25,-0.95; 3 1.25,0
SOT23 = smd 1 x 1.4: 1 -0.95,-1.1; 2 0.95,-1.1; 3 0,1.1
CT3151V1 = drill 1.7: 1 -2.38,0; 2 2.38,0; 3 0,2.38; 4 0,-2.38
_0603 = smd 0.9 x 0.8: 1 -0.762,0; 2 0.762,0
TBC05031GG = drill 1.3 pad 1.95 square: 1 0,0 | drill 1.3 pad 1.95: 2 2.54,0; 3 5.08,0
HE3621A0500 = drill 0.8 pad 1.3: 1 0,0; 2 5.08,0; 3 10.16,0; 4 15.24,0
LQM21PHR47NG0D = smd 1.15 x 1: 1 -1.175,0; 2 1.175,0
INDC3225X270N = smd 1.3 x 2.7: 1 -1.4,0; 2 1.4,0
INDC2012X145N = smd 1.2 x 1.45: 1 -0.85,0; 2 0.85,0
2PINHEADER = drill 1 long: P0 -1.27,0; P1 1.27,0
6PINHEADER = drill 1 long: P0 1.27,-1.778; P1 3.81,-1.778; P2 6.35,-1.778; P3 8.89,-1.778; P4 11.43,-1.778; P5 13.97,-1.778
CHIPLED_0603 = smd 0.8 x 0.8: A 0,-0.75; C 0,0.75
SOT23-R = smd 0.635 x 1.016: 1 -0.95,-1; 2 0.95,-1; 3 0,1
R0603 = smd 1 x 1.1: 1 -0.85,0; 2 0.85,0
R1206 = smd 1.6 x 1.803: 1 -1.422,0; 2 1.422,0
LVK12R100CER = smd 1.75 x 1.1: 1 -1.375,0.7; 2 1.375,0.7; 3 -1.375,-0.7; 4 1.375,-0.7
SHORT_TOP-50 = smd 1.27 x 1.27: 1 0.635,0; 2 -0.635,0
SOP65P640X120-28N = smd 1.475 x 0.45: 1 -2.938,4.225; 2 -2.938,3.575; 3 -2.938,2.925; 4 -2.938,2.275; 5 -2.938,1.625; 6 -2.938,0.975; 7 -2.938,0.325; 8 -2.938,-0.325; 9 -2.938,-0.975; 10 -2.938,-1.625; 11 -2.938,-2.275; 12 -2.938,-2.925; 13 -2.938,-3.575; 14 -2.938,-4.225; 15 2.938,-4.225; 16 2.938,-3.575; 17 2.938,-2.925; 18 2.938,-2.275; 19 2.938,-1.625; 20 2.938,-0.975; 21 2.938,-0.325; 22 2.938,0.325; 23 2.938,0.975; 24 2.938,1.625; 25 2.938,2.275; 26 2.938,2.925; 27 2.938,3.575; 28 2.938,4.225
R_8_ADI-L = smd 1.876 x 0.508: 1 -2.613,1.905; 2 -2.613,0.635; 3 -2.613,-0.635; 4 -2.613,-1.905; 5 2.613,-1.905; 6 2.613,-0.635; 7 2.613,0.635; 8 2.613,1.905
SOT95P280X125-5N = smd 1.2 x 0.55: 1 -1.25,0.95; 2 -1.25,0; 3 -1.25,-0.95; 4 1.25,-0.95; 5 1.25,0.95
SOT65P210X110-5N = smd 1.2 x 0.4: 1 -0.95,0.65; 2 -0.95,0; 3 -0.95,-0.65; 4 0.95,-0.65; 5 0.95,0.65
SOP65P490X110-8N = smd 1.4 x 0.45: 1 -2.2,0.975; 2 -2.2,0.325; 3 -2.2,-0.325; 4 -2.2,-0.975; 5 2.2,-0.975; 6 2.2,-0.325; 7 2.2,0.325; 8 2.2,0.975
SOP65P640X100-21N = smd 1.475 x 0.4: 1 -2.938,2.925; 2 -2.938,2.275; 3 -2.938,1.625; 4 -2.938,0.975; 5 -2.938,0.325; 6 -2.938,-0.325; 7 -2.938,-0.975; 8 -2.938,-1.625; 9 -2.938,-2.275; 10 -2.938,-2.925; 11 2.938,-2.925; 12 2.938,-2.275; 13 2.938,-1.625; 14 2.938,-0.975; 15 2.938,-0.325; 16 2.938,0.325; 17 2.938,0.975; 18 2.938,1.625; 19 2.938,2.275; 20 2.938,2.925 | smd 2.4 x 4: 21 0,0
3PINHEADER = drill 1 long: N0 1.27,1.27; N1 3.81,1.27; N2 6.35,1.27
2PINHEADER_S = drill 1 pad 1.778: N0 2.59,0.056; N1 0.05,0.056
1PINHEADER_S = drill 1 pad 1.778: P$1 1.27,1.27

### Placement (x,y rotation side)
C1  41.5,17.75 0 top
C2  42.95,14.4 270 top
C3  51.9,22.1 90 top
C4  45.2,20.45 270 top
C5  53.19,1.63 0 top
C6  40.59,3.88 0 top
C7  54.05,28.55 90 top
C8  40.65,28.6 270 top
C9  52.05,29.1 90 top
C10  40.59,8.01 0 top
C11  40.57,5.95 0 top
C12  48.81,4.96 270 top
C13  46.78,5.26 270 top
C14  44.75,5.56 270 top
C15  53.68,13.95 180 top
C16  36.97,13.29 90 top
C17  23.8,33.35 180 top
C18  56.88,12.78 0 top
C19  59.82,8.02 270 top
C20  25.62,29.08 270 top
C21  36.46,22.63 270 top
C22  23.57,27.82 90 top
C23  33.8,19.88 270 top
C24  40.67,24.18 270 top
C25  29.48,18.66 180 top
C26  33.2,36.95 90 top
C28  62.82,39.35 0 top
C29  59.48,39.4 180 top
C32  58.43,60.95 180 top
C33  62.52,61 0 top
C34  24.13,38.1 180 top
C35  30.42,38.1 0 top
C38  60.9,37.1 180 top
C40  27.3,38.1 0 top
C41  60.3,58.65 0 top
C44  31.25,20.75 180 top
C45  38.55,24.2 270 top
C46  42.65,28.7 270 top
C47  31,6.7 0 top
C48  27.8,6.7 180 top
C49  55.45,20.4 270 top
C50  46.2,15.55 0 top
D1  48.68,8.7 0 top
D2  41.69,10.14 180 top
D3  37.95,36.85 90 top
D4  57.2,50.85 90 top
D5  24.75,8.15 90 top
D6  8.3,32.25 270 top
D7  3.4,32.3 270 top
D8  13,32.4 270 top
DCI1  73.5,55 0 top
DCI2  73,36 0 top
FB1  31.3,13.25 180 top
J1  25.9,81 0 top
J2  61.97,81 0 top
J3  82.89,48 270 top
K1  9.65,62 0 top
K2  9.65,54.5 0 top
K3  9.65,47 0 top
K4  47.15,61.1 180 top
K5  47.15,53.6 180 top
K6  47.15,46.1 180 top
L1  50.76,8.16 270 top
L2  36.97,9.26 270 top
L3  57.6,20.35 270 top
L4  45.75,12.75 270 top
N1  84,63.5 90 top
N2  63.7,45.5 90 top
N3  23.2,5.3 0 top
N4  7.94,5.3 0 top
N5  5.38,3.51 0 top
PWR  4.05,13 0 top
Q1  11.25,24.85 0 top
Q2  9.1,19.85 0 top
Q3  11.1,28.35 0 top
R1  52.37,16.04 0 top
R2  50.62,13.94 180 top
R3  50.63,11.83 0 top
R4  10.52,15.42 90 top
R5  53.68,11.66 0 top
R6  13.25,15.42 90 top
R7  15.93,15.42 90 top
R8  4.35,24.7 0 top
R9  18.66,15.47 90 top
R10  21.39,15.47 90 top
R11  26.02,17.47 90 top
R12  15.39,9.82 90 top
R13  21.33,12.08 270 top
R14  27.82,14.7 0 top
R15  7.83,8.72 90 top
R16  10.27,12.59 0 top
R17  7.75,23.75 90 top
R18  4.35,19.75 0 top
R19  62.8,41.55 180 top
R20  59.45,41.55 0 top
R21  4.4,17.3 0 top
R22  4.1,28.3 0 top
R23  59,63.8 270 top
R24  62,63.9 270 top
R25  24.95,40.6 270 top
R26  30.15,40.65 270 top
R27  7.7,28.1 90 top
R28  5.15,58 90 top
R29  5.15,49 90 top
R30  4.25,41.3 0 top
R31  51.55,58.2 90 top
R32  51.55,49 90 top
R33  51.55,41.1 90 top
R34  4.9,9.55 0 top
R35  68.2,45.6 90 top
SENSE+  55,72 0 top
SENSE-  74,72 0 top
SH2  43.1,5.2 0 bottom
U1  31.45,26.99 0 top
U2  47.31,28.95 180 top
U3  48.56,22.26 180 top
U4  40.05,15.25 180 top
U5  28.8,34.85 0 top
U7  55.24,6.59 270 top
U$1  42.7,81 0 top
U$2  32.65,9.45 180 top
U$3  16.75,37.11 0 top
U$4  61.58,19.45 0 top
U$6  3.85,51.4 0 top
U$7  65.5,48.85 0 top
U$8  3.85,42.6 0 top
U$9  26.26,8.15 0 top
U$11  50.25,51.7 0 top
U$12  50.25,42.9 0 top
U$13  65.5,39.95 0 top
VIN+  19,72 0 top
VIN-  38,72 0 top

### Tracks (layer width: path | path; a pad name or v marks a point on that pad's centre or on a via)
A2
  Top 0.305: U1.23 35.76,27.96 40.55,32.75 58.5,32.75 61.75,36 C38.1
  Top 0.813: R19.2 61.95,39.37 C28.1 61.97,37.32 C38.1
A3
  Top 0.305: U1.24 35.66,28.61 40.3,33.25 56.2,33.25 C38.2
  Top 0.813: R20.2 60.3,39.43 C29.1 60.33,37.38 C38.2
A5
  Top 0.305: U1.26 36.26,29.91 40.25,33.9 54.95,33.9 57.1,36.05 57.1,44.4 61.2,48.5 61.2,58.6 C41.2
  Top 1.016: R24.2 61.67,62.72 C33.1 61.67,59.17 C41.2
A6
  Top 0.254: 59.3,60.97 C32.1 | 54.5,34.45 56.4,36.35 56.4,38.8
  Top 0.305: U1.27 36.16,30.57 40.05,34.45 54.5,34.45 | 56.4,38.8 56.4,44.6 59.45,47.65 C41.1
  Top 1.016: R23.2 59.28,62.67 C32.1 59.28,58.82 C41.1
A7
  Top 0.254: 34.34,31.27 U1.28 35.76,31.21 39.7,35.15 54.05,35.15 55.8,36.9 55.8,49.15 D4.1
A8
  Top 0.406: C34.1 24.98,35.32 25.77,34.52 U5.3
  Top 0.813: 25,38.12 C34.1 | 26.48,38.13 C40.1
  Top 1.016: R25.2 24.95,38.13 C34.1 C40.1 26.46,38.09
A8_BUF
  Top 0.406: U5.1 27.67,35.83 28.51,34.99 U1.1
  Top 0.508: U5.1 U5.2
A9
  Top 0.305: C40.2 29.3,38.1
  Top 0.406: 29.3,38.1 29.3,34.55 29.97,33.88 U5.5
  Top 0.813: 29.6,38.13 C35.1 | 28.17,38.12 C40.2
  Top 1.016: R26.2 29.6,39.25 29.6,38.13 | C35.1 28.19,38.1 28.17,38.12
A9_BUF
  Top 0.406: U1.2 30.66,30.57 32.65,32.55 32.65,34.45 31.92,35.17 U5.7
  Top 0.508: U5.7 U5.6
ACOM
  Top 0.305: U1.3 31.56,29.91 37,35.35
  Top 0.406: 37,35.35 D3.1
AGND  (via drill 0.3)
  Top 0.406: U1.25 32.66,29.27 v32.6,29.2 | U1.22 32.63,27.32 v32.6,27.35
  Top 0.508: U2.4 49.92,31.52 v50.15,31.75 | C9.2 52.05,31.05 v51.95,31.15 | C7.2 54.05,30.4 v53.9,30.55 | C8.2 40.65,26.65 v40.6,26.6 | C46.2 42.65,26.7 v42.6,26.65 | C34.2 23.18,38 v22.05,38 | C35.2 31.8,38.63 v31.8,39.7 | C26.2 v33.2,39.15 | C17.2 22.9,33.3 v21.7,33.3 | C32.2 57.58,59.38 v57.55,59.35 | C33.2 63.37,59.47 v63.3,59.4 | C29.2 58.63,37.93 v58.45,37.75 | C28.2 64.85,39.35 v64.95,39.25 | R33.1 v51.55,38.9 | R30.1 v2,41.3
  other vias: 20.25,27.25 30.4,28.75 58,33.75 40,50.25 41.5,37.75 11.75,49.25 82,34.75 82.25,28.5 71.75,30.95 58.4,28.1 53,52.75 58,47.75 63.25,49 61.1,43.2 73.25,45.75 60.3,54.45 60.55,66.4 79.4,63.2 83.1,52.65 69.55,57.65 77.7,69.25 46.25,74.6 44.45,51.4 68.5,38.15 27.45,41.15 17.55,29.9 3.1,53 2.85,44.3 2.6,59.9 19.45,58.2 28.25,61.05 28.55,68 7,69.65 13.65,73.85 11.7,57.65 39.45,61.35 28.05,54.2 51.9,62.8 42.05,69.85 54.7,81.5 46.8,78.7 38.1,82.45 34.6,75.15 28.2,75 22.9,76.05 19.4,82.15 11.3,81.4 78.05,83.1 84.1,75.2 64.85,74.8 5.6,78.5 22.6,61.9 45.8,66.55 34.8,54.75 47.2,38.2
  pour Bottom (isolate 0.5): -1.75,37 15.75,37 16.5,36.25 16.5,26 88.75,26 88.75,87.5 88.5,87.75 -0.75,87.75 -1.75,86.75
  pour Route2 (isolate 0.305): -3.14,23 88.25,23 88.25,87 88,87.25 -1,87.25 -3.14,85.11
  pour Top (isolate 0.5): -3.25,37 15.5,37 16.5,36 16.5,26 88.25,26 88.25,68.75 88,69 88,87.25 -1.5,87.25 -2.5,86.25 -2.5,41.25 -3.25,40.5
AIN2
  Top 0.813: R35.1 N2.P0 63.7,41.6 R19.1
AIN3
  Top 0.813: R35.2 67.29,46.77 N2.P1 61.87,46.77 58.6,43.5 R20.1
AIN5
  Top 0.406: R24.1 69.25,72
  Top 1.016: J2.3 74,75.41 SENSE-.3 | SENSE-.3 SENSE-.1 | SENSE-.1 SENSE-.4 SENSE-.2 SENSE-.3 | 69.25,72 SENSE-.1
  Top 1.27: SENSE-.2 SENSE-.1 | SENSE-.3 SENSE-.4
AIN6
  Top 1.016: J2.1 61.97,81.35 SENSE+.3 | SENSE+.3 SENSE+.1 SENSE+.4 | SENSE+.4 SENSE+.2 SENSE+.3 | SENSE+.4 59,65.62 R23.1
  Top 1.27: SENSE+.2 SENSE+.1 | SENSE+.3 SENSE+.4
AIN8
  Top 1.27: K1.4 K2.4 K3.4 24.95,46.94 R25.1
AIN9
  Top 1.27: K4.4 K5.4 K6.4 30.15,44.34 R26.1
CIPO
  Top 0.2: 21.33,14.56 R10.1
  Top 0.254: 21.33,14.56 R13.1 21.87,12.93 23.6,11.2 23.6,4.39 N3.P0
COPI
  Top 0.254: R9.1 18.66,11.04 21.91,7.79 N4.P5
CS
  Top 0.2: R6.1 13.25,10.7 14.98,8.97 R12.1 16.83,7.53 N4.P3
CTRL_2V
  Top 0.152: N5.P0 1.7,5.92 1.7,18.05 R18.1
CTRL_20V  (via drill 0.35)
  Top 0.152: v1.85,23.35 2.05,23.35 R8.1
  Bottom 0.152: N5.P1 1.85,8.31 v1.85,23.35
CTRL_200V  (via drill 0.35)
  Top 0.152: v2.8,26.55 2.8,27.95 R22.1
  Bottom 0.152: N4.P0 5.1,7.63 5.1,24.1 2.8,26.4 v2.8,26.55
DCI_NEG
  Top 0.254: R35.4 68.9,47.99 U$7.P$1
  Top 1.016: 72.97,52.62 DCI1.4
  Top 1.15: R35.4 68.9,48.55
  Top 1.27: 68.9,48.55 72.97,52.62 | J3.1 78.12,48 DCI1.4 | DCI1.1 DCI1.3 DCI1.2 | DCI1.1 DCI1.4 | DCI1.4 DCI1.2 | DCI1.1 DCI1.2
DCI_POS
  Top 0.254: U$13.P$1 68.9,43.35 R35.3
  Top 1.15: R35.3 68.9,42.48
  Top 1.27: 68.9,42.48 DCI2.3 | J3.3 77.54,42.92 DCI2.3 | DCI2.3 DCI2.1 | DCI2.1 DCI2.4 DCI2.2 | DCI2.2 DCI2.3 | DCI2.1 DCI2.2
DRDY  (via drill 0.35)
  Top 0.2: R11.1 25.67,16.27 25.67,13.88 v25.77,13.78 26.47,14.47 26.82,14.47 26.97,14.62 R14.1
  Route15 0.2: v25.77,13.78 25.77,4.76 N3.P1
GND  (via drill 0.3, 0.35)
  Top 0.254: U7.19 57.51,2.04 v57.65,1.9
  Top 0.508: C45.2 38.55,22.05 38.28,21.78 | 38.28,21.78 v38.25,21.75 | C24.2 40.67,22.97 v39.55,21.85 | C21.2 38.28,21.78 | C4.2 46.6,19.6 v46.65,19.65 | 50.95,22.3 50.91,22.26 U3.2 51.21,22.26 C3.2 | C3.2 v51.9,24.35 | C3.2 v53.3,22.95 | C49.2 55.4,19.5 v53.95,19.5 | D5.P$1 v24.75,7.15 25.2,6.7 C48.2 | C47.2 v33.05,6.7 | v42.75,10.45 42.7,10.4 41.95,10.4 D2.P$1 41.44,9.89 C10.2 41.42,7.99 C11.2 41.44,5.93 C6.2 v41.45,2.3 | C25.2 28.34,18.66 v27.55,19.45 | C23.2 34.87,19.03 v35.3,18.6 | C1.2 43.7,17.75 v43.75,17.7 | C2.2 42.85,13.45 v41.3,13.45 41.3,14.3 U4.1 | C16.2 35.46,14.14 v35.4,14.2 | C50.2 47.05,16.7 v47.65,17.3
  Route15 0.254: v57.65,1.9 58.05,2.3 v58.05,15.35
  Bottom 0.508: SH2.1 39.9,5.2 39.1,6 36.21,6 34.63,4.42 N3.P4
  other vias: 36.55,24.65 11.2,18.85 23.3,15.55 24.4,24.5 25.15,19.7 58.15,23.1 7.7,26.1 13.1,27.4 1.7,30.15 14.85,30.75 12.2,22.7 74.75,18.4 84.55,23.4 65.59,7.47 84.55,17.87 65.5,2.45 66.23,18.23 74.83,23.83 85.05,8.4 79.05,1.4 60.95,17.2 7.7,21.75 3.1,22.6 17.5,12.95 3.55,15.75 7.1,12.55 5.7,13.65 2.55,6.55 5.3,6.4 12.65,8.1 15,7.4 18.25,7.6 20.55,7.6 23.75,13.1 30.65,16.75
  pour Top (isolate 0.254): -1.45,0.3 -1.45,25.3 63.65,25.3 64.2,24.75 64.2,15.2 63.8,14.8 48.15,14.8 42.75,9.4 42.75,-2 0.85,-2
  pour Bottom (isolate 0.254): 24.25,-1 -1,-1 -1,25.5 63.4,25.5 63.9,25 63.9,15.15 63.5,14.75 48.1,14.75 42.8,9.45 42.8,0 40.05,-2.75 26,-2.75
  pour Route2 (isolate 0.254, no thermals): -2.25,12.25 -2.25,25.5 63.5,25.5 64.05,24.95 64.05,15.35 63.45,14.75 48.1,14.75 42.8,9.45 42.8,-1 42.3,-1.5 -1.25,-1.5 -2,-0.75 -2,12
  pour Bottom (isolate 0.254): -3,24.25 -3,36.25 15.25,36.25 16,35.5 16,25 15.25,24.25
  pour Route2 (isolate 0.254): -4,24.25 -4,36.25 15.25,36.25 16,35.5 16,24.25
  pour Top (isolate 0.254): -3.75,23.5 -3.75,35.5 -3,36.25 15.25,36.25 16,35.5 16,24 -3.25,24
  pour Bottom: 63.75,-0.75 63.75,15.5 63.75,20.75 63.75,25.25 88.25,25.25 88.25,11.75 88.25,-0.75 87.5,-1.5 64.5,-1.5
  pour Route2: 63.75,-1.75 63.75,16.5 63.75,25.25 88.5,25.25 88.5,9 88.5,-1 87.75,-1.75
  pour Top: 63.75,-2.5 63.75,19.25 63.75,25.25 88.75,25.25 89,25 89,16.25 89,-1 88.75,-1.25 87.75,-2.25 86.5,-2.25 64,-2.25
IDAC1
  Top 0.254: D3.3 40.25,35.8 53,35.8 54.85,37.65 54.85,48.05 54.3,48.6 54.3,63.7 43.97,74.03 U$1.N0
IDAC2
  Top 0.254: D4.3 55.25,54.05 55.25,64.25 49.1,70.4 49.1,82.28 U$1.N2
N$2
  Top 0.152: R8.2 R17.2 9.45,24.7 Q1.1
N$4
  Top 0.254: 53.61,10.88 R5.1 C15.2
  Top 0.305: U7.8 53.61,10.88 | R3.2 52.66,11.83 R5.1
N$5
  Top 0.508: 50.95,9.53 U7.10
  Top 0.61: 50.95,9.53 L1.1
  Top 0.813: L1.1 48.69,9.34 D1.1
N$6
  Top 0.305: U7.7 54.26,11.39 R5.2 55.65,12.78 C18.1
N$7
  Top 0.305: C15.1 54.53,14.55 53.22,15.86 R1.2
N$8
  Top 0.254: U1.4 26.83,29.27 26.16,29.93 C20.1
N$9
  Top 0.254: U1.5 27.35,28.61 26.97,28.23 C20.2
N$10
  Top 1.27: R28.1 7.57,56.58 K2.1 7.82,52.67 U$6.P$1 5.12,50.45 R29.2
N$11
  Top 0.254: R3.1 49.78,12.18 50.45,12.85 51,12.85 51.47,13.32 R2.1
N$12
  Top 0.813: 5.12,41.37 R30.2
  Top 1.27: R29.1 5.73,47 K3.1 6.52,43.87 U$8.P$1 5.12,41.37
N$14
  Top 1.27: R31.1 50.33,56.78 K5.1 47.78,52.97 U$11.P$1 51.55,52.94 R32.2
N$16
  Top 1.27: R32.1 48.63,47.58 K6.1 49.08,44.17 U$12.P$1 51.55,44.14 R33.2
N$17
  Top 0.508: U$2.N0 30.06,9.49 31.01,10.44 31.01,10.45 31.66,11.1 31.66,12.85 FB1.1
N$19
  Top 0.2: R34.1 PWR.A
N$22
  Top 0.152: Q2.1 7.25,19.75 R18.2 5.3,17.25 R21.2
N$25
  Top 0.152: R22.2 6.95,28.3 R27.2 8.45,29.05 Q3.1
N$28
  Top 0.254: U1.17 35.87,24.07 C21.1
PE  (via drill 0.3)
  Bottom 0.508: SH2.2 46.38,7.85 v46.4,7.85
  other vias: 56.65,1.4 53.85,7.3 55.1,7.3 56.35,7.3 53.85,6.05 55.1,6.05 56.35,6.05 60.45,13.55 50.7,3.65 60.15,4 45.1,2.3 52.5,5.9 52.4,7.15 46.35,10.1
  pour Bottom (no thermals): 62.8,14.3 48.85,14.3 43.6,9.05 43.6,-0.95 61.8,-0.95 63.05,0.3 63.05,14.05
  pour Route2 (no thermals): 43.55,-2 43.55,8.95 47.05,12.45 47.05,12.5 48.8,14.25 63.25,14.25 63.25,-0.75 62.5,-1.5 44.05,-1.5
  pour Top (no thermals): 43.55,-2.75 43.55,9 48.8,14.25 63.15,14.25 63.15,-1.1 62.25,-2 44.3,-2
RNG_2V  (via drill 0.35)
  Top 0.254: v9.65,22.05 9.65,21.4 Q2.3
  Top 0.508: v2.9,34.35 2.3,33.75 D7.1
  Route15 0.406: v2.9,34.35 4.95,36.4 9.45,36.4 13.45,40.4 13.45,55.47 14.27,56.46 K1.3
  Bottom 0.254: v2.9,34.35 3,34.25 3,28.7 v9.65,22.05
  Bottom 0.508: K4.3 34.91,57.9 22.75,57.9 K1.3
RNG_20V  (via drill 0.35)
  Top 0.254: v12.45,25.95 12.35,25.85 Q1.3
  Top 0.508: v7.5,34.4 7.2,34.1 D6.1
  Route15 0.406: v7.5,34.4 8.55,35.45 10.35,35.45 16.95,42.05 16.95,49.34 K2.3
  Route15 0.508: 7.55,34.4 v7.5,34.4
  Bottom 0.254: v7.5,34.4 7.5,33.15 12.45,28.2 v12.45,25.95
  Bottom 0.508: K5.3 36.5,53.6 35.12,52.22 23.34,52.22 21.06,54.5 K2.3
RNG_200V  (via drill 0.35)
  Top 0.254: v12.25,29.95 11.7,29.95 Q3.3
  Top 0.508: v11.85,34.6 11.9,34.55 D8.1
  Bottom 0.254: v11.85,34.6 11.95,34.5 11.95,30.25 v12.25,29.95
  Bottom 0.508: v11.85,34.6 11.81,34.64 11.81,35.7 K3.3 22.2,44.75 34.72,44.75 35.98,45.09 K6.3
RST  (via drill 0.35)
  Top 0.152: N4.P1 7.83,7.44 R15.1
  Top 0.2: U1.20 33.36,26.02 32.35,25 v32.25,25 | U7.3 56.86,11.04 56.85,11.05 v56.8,11.05
  Route15 0.2: v32.25,25 32.25,22.75 25.5,16 | 25.5,16 24.1,14.6 15.5,14.6 11.65,10.75 11.65,3.62 N4.P1 | v56.8,11.05 52.15,15.7 25.8,15.7 25.5,16
SCLK
  Top 0.254: R7.1 15.93,12.52 19.37,9.08 N4.P4
START
  Top 0.2: 11.15,12.56 R16.2 | R4.1 11.12,13.97 R16.2 | R16.2 11.12,11.53 13.85,8.8 13.85,3.96 N4.P2
UCIPO
  Top 0.254: R10.2 21.39,17.19 27.61,23.41 U1.13
UCOPI
  Top 0.254: R9.2 19.84,17.5 20.85,17.5 27.41,24.07 U1.12
UCS
  Top 0.2: R6.2 15.53,18.55 20.55,18.55 27.36,25.36 U1.10
UDRDY
  Top 0.2: R11.2 26.02,20.27 U1.14
USCLK
  Top 0.254: R7.2 17.81,18.15 20.7,18.15 27.26,24.71 U1.11
USTART
  Top 0.2: R4.2 13.2,18.95 20.45,18.95 27.51,26.02 U1.9
V+  (via drill 0.35)
  Top 0.254: U1.6 29.83,27.96 31.2,26.6 31.2,22.4 32.12,21.48 | U3.5 | 32.24,20.73 32.12,20.85 | 35.9,19.45 35.9,20.15 35.95,20.2 v35.85,20.3 | v33.45,34.9 33.45,35.85 C26.1 32.92,35.83 U5.8
  Top 0.305: 32.12,21.48 32.12,20.85 32.12,20.73 C44.1
  Top 0.406: U3.5 C4.1 43.35,19.45 35.9,19.45 35.53,19.45 34.25,20.73 C23.1 32.24,20.73
  Bottom 0.254: v35.85,20.3 33.35,22.8 33.35,32.45 33.45,32.55 v33.45,34.9
V-  (via drill 0.35)
  Top 0.2: C22.2 23.57,28.48
  Top 0.254: 30.58,18.41 30.34,18.64 C25.1 | 23.57,28.48 24.73,27.32 U1.7 29.48,27.32 30.43,26.37 30.4,26.34 C44.2 | 41,17.4 C1.1 40.35,17.45 | 31.8,17.45 31.75,17.5 31.75,18.3 v31.8,18.35 | v24.65,31.75 C17.1 25.17,33.88 U5.4
  Top 0.305: 30.2,18.5 30.34,18.64 | 30.33,20.68 C44.2
  Top 0.406: C25.1 30.33,20.68 | U4.3 41,17.4 | 30.2,18.5 31.25,17.45 31.8,17.45 40.35,17.45
  Bottom 0.254: v31.8,18.35 29.6,20.55 29.6,26.8 v24.65,31.75
VCC  (via drill 0.35)
  Top 0.406: C16.1 37.03,12.4
  Top 0.61: L2.1 36.86,10.77 C16.1 | v57.1,17.75 57.6,18.25 L3.2 | 37.03,12.4 v38.95,12.4
  Bottom 0.406: 57.1,17.65 v57.1,17.75
  Bottom 0.61: v38.95,12.4 44.1,12.4 48.55,16.85 56.3,16.85 57.1,17.65
VCC_LP  (via drill 0.35)
  Top 0.152: U3.3 49.01,23.21 48.5,22.7 48.5,21.6 48.79,21.31 U3.1 49.81,20.41 v49.15,19.75 | v37.6,16.7 38.3,16.7 U4.4
  Top 0.254: C49.1 54.95,21.75 54.95,26.8 C7.1 | U2.2 49.91,28.25
  Top 0.305: C3.1 49.87,21.25 U3.1 | D7.3 4.75,32.55 v4.75,33.75 6.3,35.3 8.1,35.3 9.4,34 | 9.4,34 D6.3 | 9.4,34 10.7,35.3 10.7,35.35 13.3,35.35 14.1,34.55 D8.3
  Top 0.406: 55.5,21.2 C49.1 C3.1 | C7.1 53.5,28.25 C9.1 49.91,28.25
  Top 0.508: C49.1 55.45,22.4 v56.25,23.2
  Top 0.61: L3.1 55.5,21.2
  Bottom 0.152: v49.15,19.75 46.05,16.65 37.6,16.65 v37.6,16.7
  Bottom 0.305: K3.2 5.75,34.72 5.75,34.55 4.95,33.75 v4.75,33.75
  Bottom 0.508: K3.2 K2.2 K1.2 16.48,63.75 39.42,63.75 K4.2 K5.2 K6.2 42.07,42.53 44.55,40.05 48.45,40.05 56.25,32.25 v56.25,23.2
VCCIO  (via drill 0.35)
  Top 0.2: 21.6,11.5 R13.2 21.25,11.15 v21.25,10.05 | v14.7,12.35 15.39,11.66 R12.2 | FB1.2 28.6,13.25 v28.3,12.95 | v29.9,14.65 28.92,14.65 28.87,14.7 R14.2 | v9.15,10.45 8.27,9.57 R15.2 5.77,9.57 R34.2
  Top 0.254: v42.9,23.25 41.12,25.03 C24.1 40.65,25.05 C45.1 38.23,25.36 U1.19 | 30.19,13.25 FB1.2 30.54,14.01 v29.9,14.65
  Bottom 0.2: v9.15,10.45 9.45,10.75 13.1,10.75 v14.7,12.35 14.75,12.3 14.9,12.45 16.65,12.45 19.05,10.05 v21.25,10.05 23,11.8 27.15,11.8 v28.3,12.95
  Bottom 0.254: v29.9,14.65 30.75,15.5 34.65,15.5 42.4,23.25 v42.9,23.25
VIN+
  Top 1.016: 37.37,74.38 VIN-.3 | VIN-.3 VIN-.2 VIN-.4 VIN-.1 VIN-.3
  Top 1.27: J1.3 30.98,81.23 37.37,74.38 | VIN-.1 VIN-.2 | VIN-.3 VIN-.4 47.15,61.97 K4.1 48.45,59.8 49.42,59.8 49.6,59.62 R31.2
VIN-
  Top 1.016: 19.57,74.38 VIN+.3 | VIN+.3 VIN+.1 VIN+.4 | VIN+.4 VIN+.2 VIN+.3 | 18.99,72.7 18.99,71.13 VIN+.4
  Top 1.27: J1.1 25.9,81.17 19.57,74.38 | VIN+.3 VIN+.4 18.77,71.12 K1.1 7.07,59.42 R28.2 | VIN+.1 VIN+.2
VIN_DIG
  Top 0.406: N3.P3 31,4.61 31,5.85 C47.1 C48.1 27.53,7.82 U$9.P$1 26.81,10.14 D5.P$2
VIN_PWR  (via drill 0.35)
  Top 0.203: v61.6,8.35 61.08,8.87 C19.1 59.16,9.53 U7.1
  Top 0.406: U7.12 U7.13
  Top 0.61: v50.4,1.39 52.1,1.39 C5.1 52.31,1.66 U7.11 U7.12 | N3.P5 37.53,3.88 C6.1 39.74,5.93 C11.1 39.72,8.01 C10.1 | C10.1 39.7,8.73 D2.P$2 | C10.1 39.49,7.86 L2.2 34.13,7.86 U$2.N1
  Bottom 0.203: v50.4,1.39 52.91,3.9 57.3,3.9 61.6,8.2 v61.6,8.35
  Bottom 0.61: N3.P5 41.72,3.52 43.92,1.32 50.4,1.32 v50.4,1.39
VREF_2.5
  Top 0.254: U1.8 23.87,26.66 C22.1
VREF_2.048  (via drill 0.35)
  Top 0.254: 42.54,29.45 C46.1 42.66,29.54 | 44.85,29.54 U2.6 | 46.9,30.05 v47,30.05
  Top 0.406: U1.21 36.76,26.66 39.55,29.45 C8.1 42.54,29.45 | 44.85,29.54 42.66,29.54 | U2.6 46.43,29.59 46.9,30.05
  Route15 0.254: 83.97,64.8 N1.P1
  Route15 0.406: v47,30.05 56.75,39.8 56.75,48.55 73,64.8 83.97,64.8
VSS
  Top 0.152: U7.9 52.96,8.66 52.5,8.2 49.6,8.2 48.85,7.45 D1.2
  Top 0.2: R2.2 49.49,13.94 47.4,11.85 45.8,11.85 L4.2
  Top 0.305: R2.2 49.77,14.44 51.37,16.04 R1.1 | 49.92,13.95 R2.2 | R2.2 49.6,13.95
  Top 0.508: C14.1 44.75,10.9 L4.2
  Top 0.813: D1.2 48.68,5.94 C12.1 48.51,6.11 C13.1 45.05,6.11 C14.1
VSS_LP
  Top 0.305: L4.1 45.35,14 C50.1 43.25,15.55 C2.1 U4.2

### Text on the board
tNames: VIN- | AGND | VIN+ | IDAC1 | IDAC2 | SENSE+ | SENSE- | AGND | AGND | VREF / 2.048V | Precision Multimeter / by Anabit LLC | AGND | DCI1 | AGND | AIN3 | AIN2 | AGND | DCI2 | GND | VDig Pwr | Vin Pwr | Precision Multimeter / V1.2 | CTRL3 | START | SCK | CIPO | GND | C:/Users/neilf/Dropbox/Anabit/CompanyMessagingBrandingGraphics/Anabit Logo Vertical - Black.bmp | CTRL1 | CTRL2 | RST | CS | COPI | RDY | GND | VDIG | VIN
bNames: Precision Analog Side | Analog Side | Digital and Pwr Side | Digital Side | Precision Multimeter / by Anabit V1.2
